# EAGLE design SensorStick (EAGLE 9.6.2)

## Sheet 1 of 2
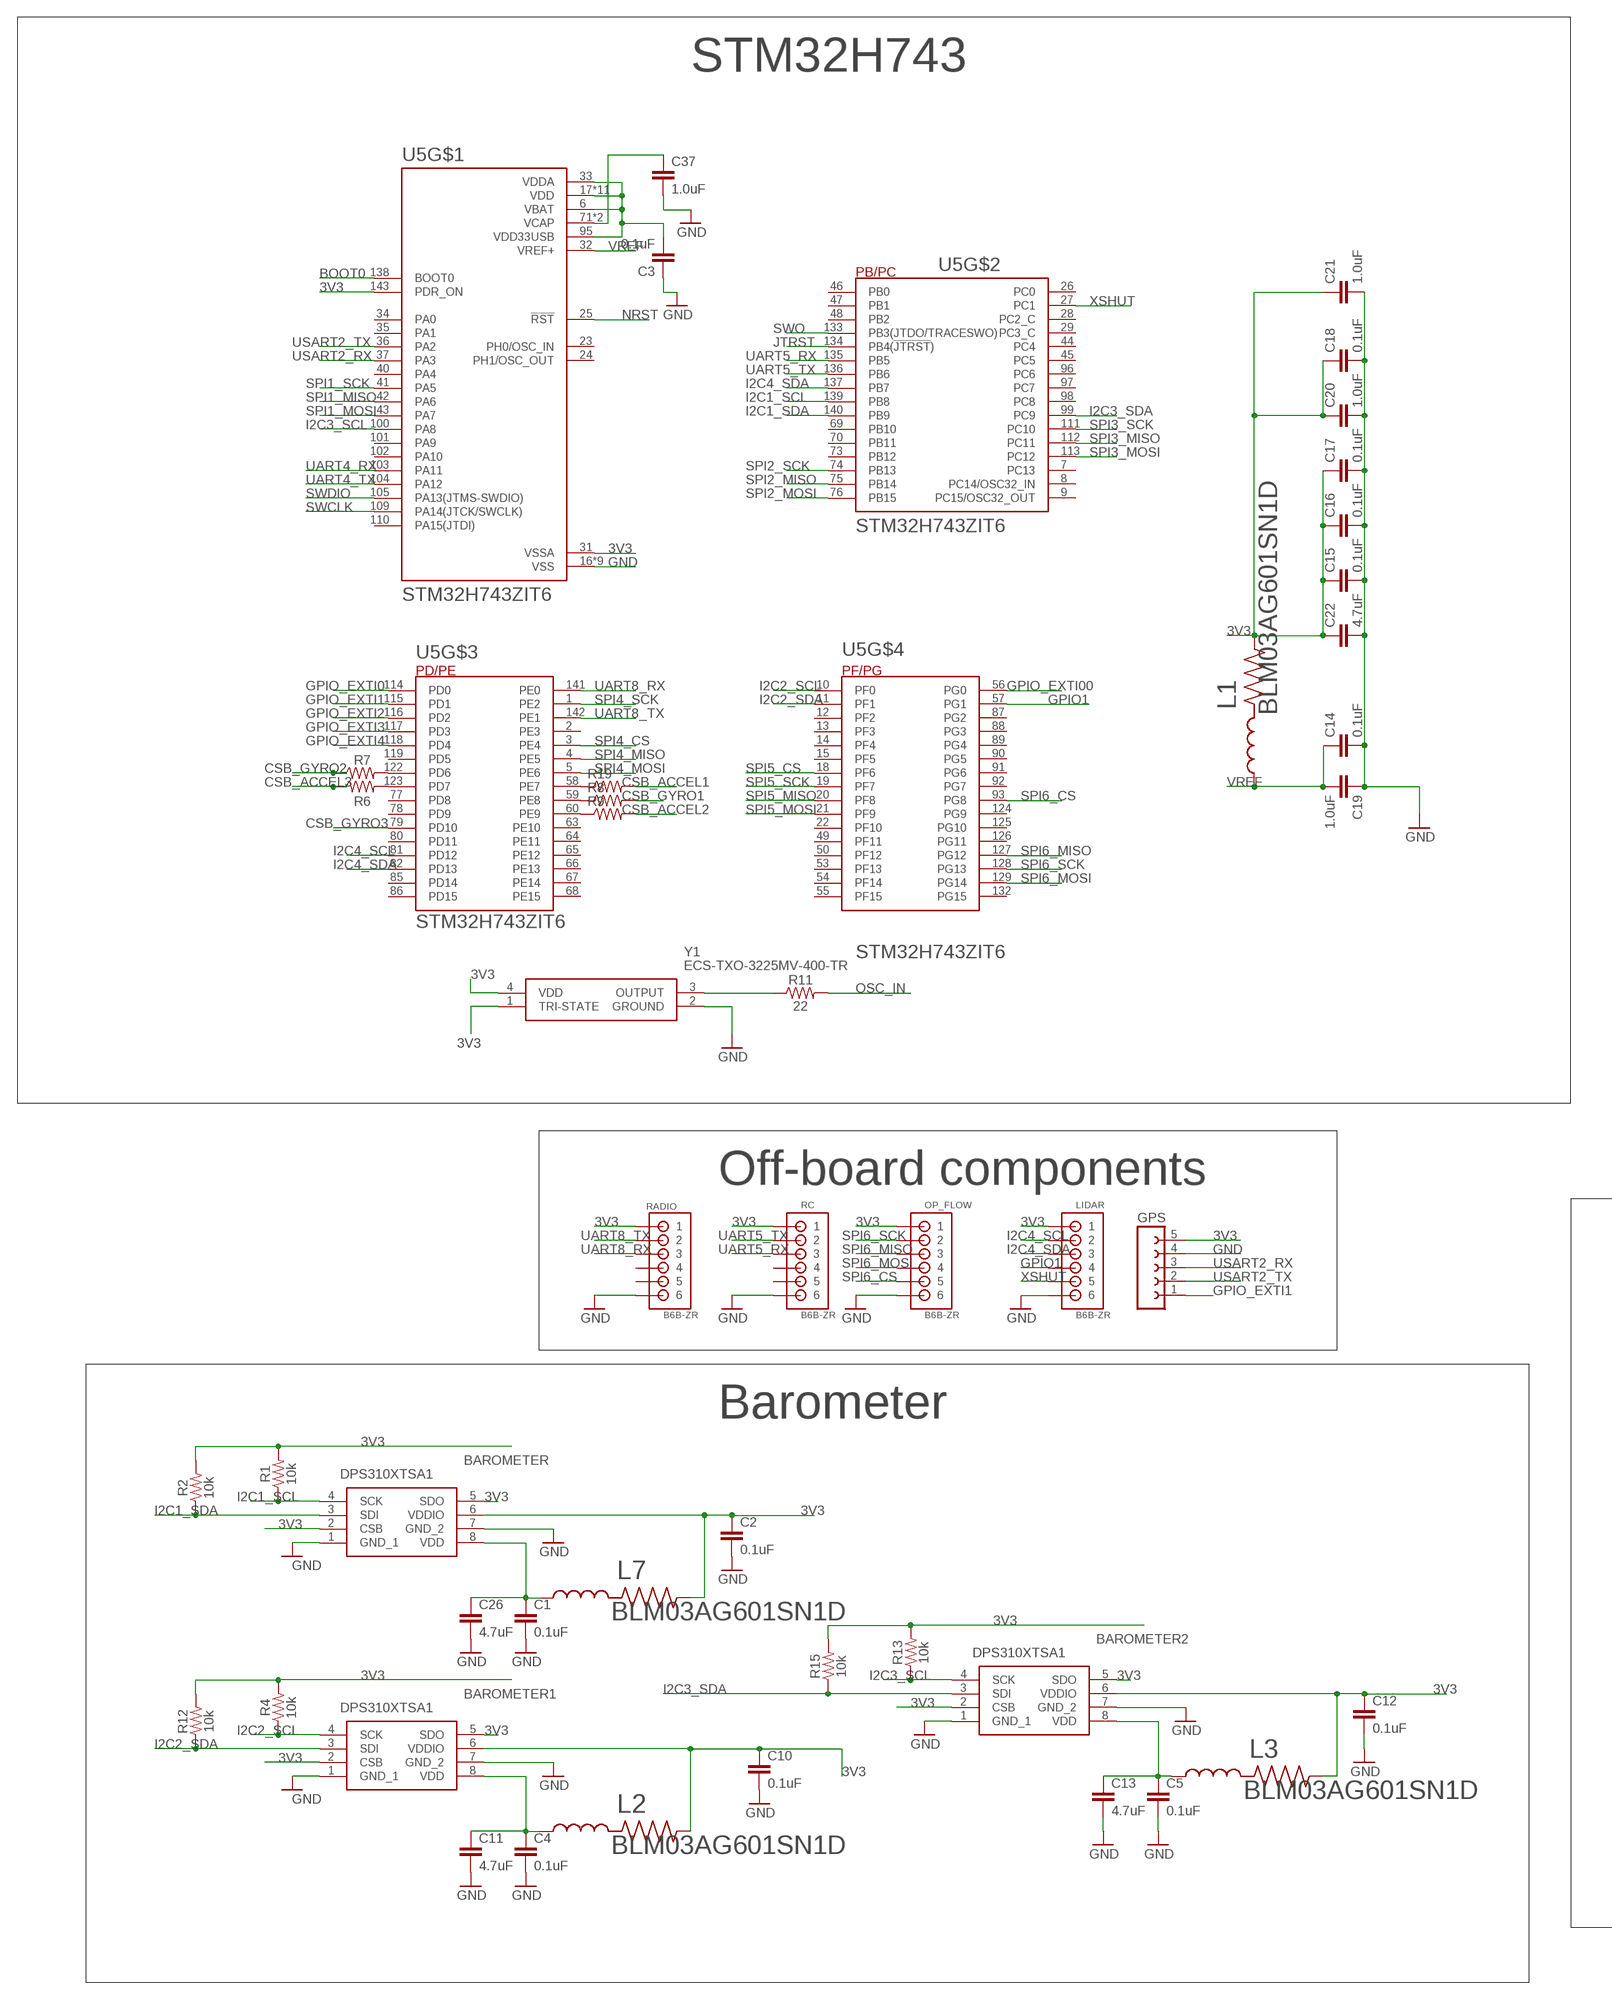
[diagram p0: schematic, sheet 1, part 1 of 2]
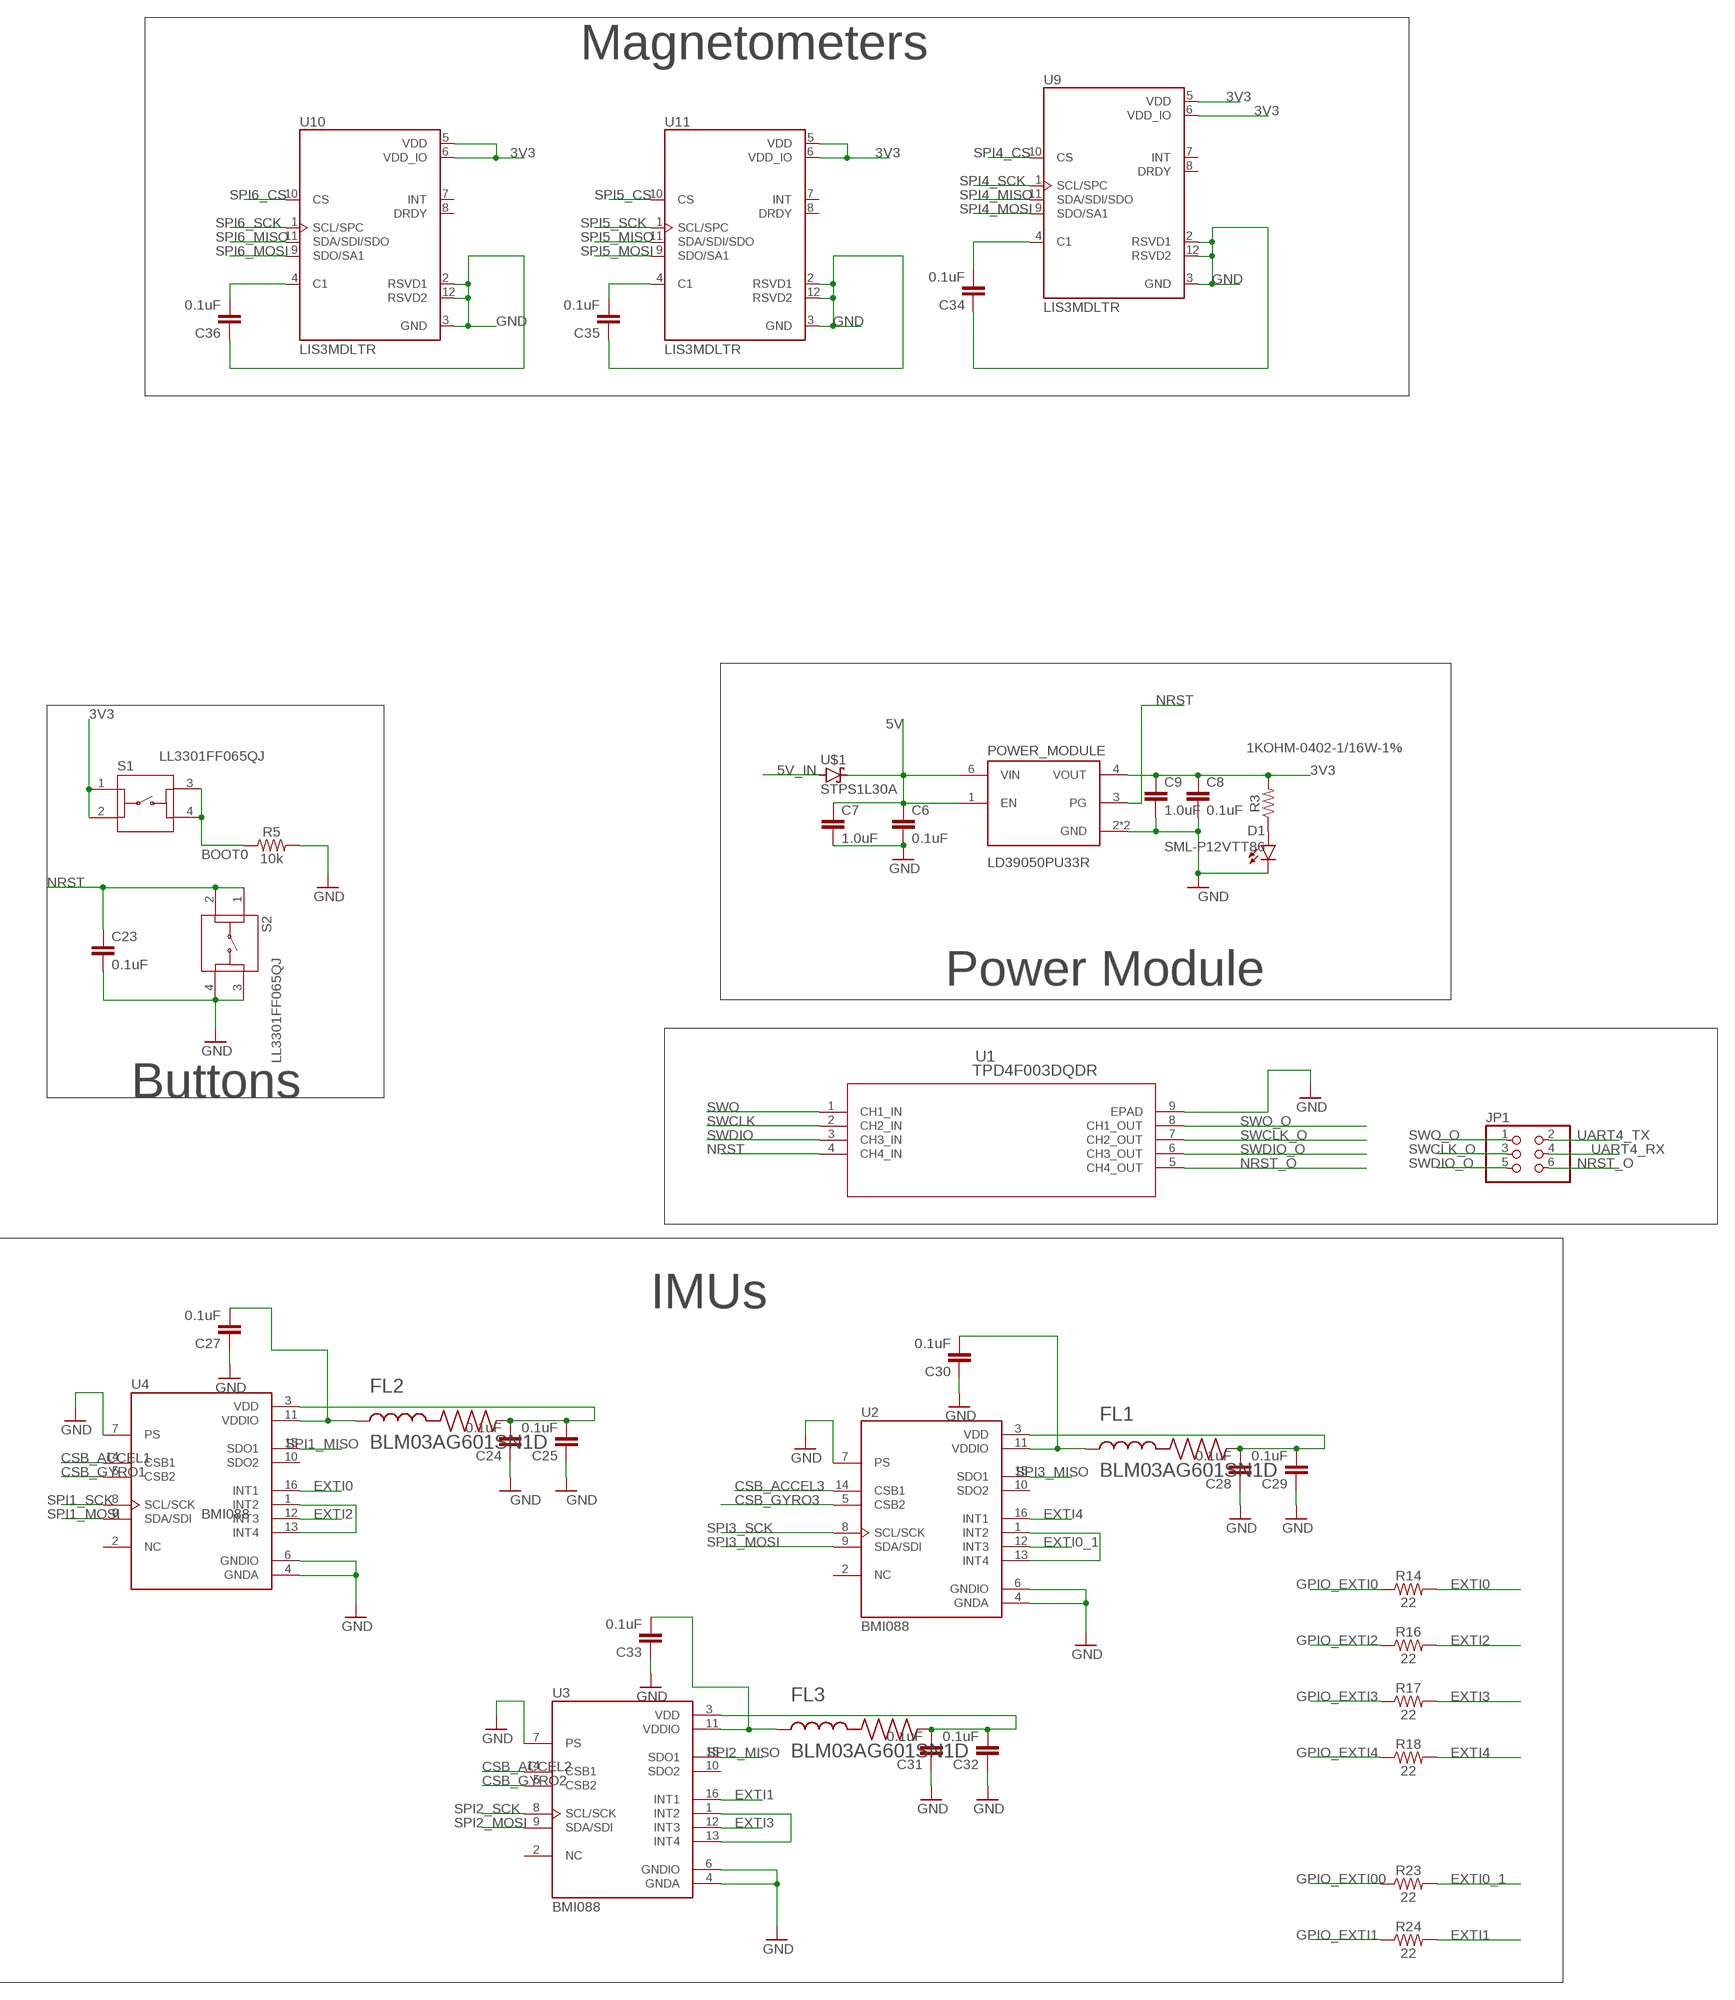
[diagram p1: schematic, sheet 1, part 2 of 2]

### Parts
BAROMETER  DPS310XTSA1  [DPS310XTSA1]
BAROMETER1  DPS310XTSA1  [DPS310XTSA1]
BAROMETER2  DPS310XTSA1  [DPS310XTSA1]
C1  0.1uF  0.1UF-0402-6.3V-10%-X7R  [0402]
C2  0.1uF  0.1UF-0402-6.3V-10%-X7R  [0402]
C3  0.1uF  0.1UF-0603-25V-5%  [0603]
C4  0.1uF  0.1UF-0402-6.3V-10%-X7R  [0402]
C5  0.1uF  0.1UF-0402-6.3V-10%-X7R  [0402]
C6  0.1uF  0.1UF-0402-6.3V-10%-X7R  [0402]
C7  1.0uF  1.0UF-0402-16V-10%  [0402]
C8  0.1uF  0.1UF-0402-6.3V-10%-X7R  [0402]
C9  1.0uF  1.0UF-0402-16V-10%  [0402]
C10  0.1uF  0.1UF-0402-6.3V-10%-X7R  [0402]
C11  4.7uF  4.7UF0603  [0603]
C12  0.1uF  0.1UF-0402-6.3V-10%-X7R  [0402]
C13  4.7uF  4.7UF0603  [0603]
C14  0.1uF  0.1UF-0603-25V-5%  [0603]
C15  0.1uF  0.1UF-0603-25V-5%  [0603]
C16  0.1uF  0.1UF-0603-25V-5%  [0603]
C17  0.1uF  0.1UF-0603-25V-5%  [0603]
C18  0.1uF  0.1UF-0603-25V-5%  [0603]
C19  1.0uF  1.0UF-0805-25V-10%  [0805]
C20  1.0uF  1.0UF-0805-25V-10%  [0805]
C21  1.0uF  1.0UF-0805-25V-10%  [0805]
C22  4.7uF  4.7UF0603  [0603]
C23  0.1uF  0.1UF-0603-25V-5%  [0603]
C24  0.1uF  0.1UF-0603-25V-5%  [0603]
C25  0.1uF  0.1UF-0603-25V-5%  [0603]
C26  4.7uF  4.7UF0603  [0603]
C27  0.1uF  0.1UF-0603-25V-5%  [0603]
C28  0.1uF  0.1UF-0603-25V-5%  [0603]
C29  0.1uF  0.1UF-0603-25V-5%  [0603]
C30  0.1uF  0.1UF-0603-25V-5%  [0603]
C31  0.1uF  0.1UF-0603-25V-5%  [0603]
C32  0.1uF  0.1UF-0603-25V-5%  [0603]
C33  0.1uF  0.1UF-0603-25V-5%  [0603]
C34  0.1uF  0.1UF-0603-25V-5%  [0603]
C35  0.1uF  0.1UF-0603-25V-5%  [0603]
C36  0.1uF  0.1UF-0603-25V-5%  [0603]
C37  1.0uF  1.0UF-0805-25V-10%  [0805]
D1  SML-P12VTT86  [LED_SML-P11UTT86R]
FL1  BLM03AG601SN1D  [BEADC0603X33N]
FL2  BLM03AG601SN1D  [BEADC0603X33N]
FL3  BLM03AG601SN1D  [BEADC0603X33N]
GPS  FE05-1  [FE05-1]
JP1  PINHD-2X3  [2X03]
L1  BLM03AG601SN1D  [BEADC0603X33N]
L2  BLM03AG601SN1D  [BEADC0603X33N]
L3  BLM03AG601SN1D  [BEADC0603X33N]
L7  BLM03AG601SN1D  [BEADC0603X33N]
LIDAR  B6B-ZR  [B6B-ZR]
OP_FLOW  B6B-ZR  [B6B-ZR]
POWER_MODULE  LD39050PU33R  [SON95P300X300X100-7N]
R1  10k  10KOHM-0402-1/16W-1%  [0402]
R2  10k  10KOHM-0402-1/16W-1%  [0402]
R3  1KOHM-0402-1/16W-1%  [0402]
R4  10k  10KOHM-0402-1/16W-1%  [0402]
R5  10k  10KOHM-0603-1/10W-1%  [0603]
R6  RT0402FRE07220RL  [RESC1005X35N]
R7  RT0402FRE07220RL  [RESC1005X35N]
R8  RT0402FRE07220RL  [RESC1005X35N]
R9  RT0402FRE07220RL  [RESC1005X35N]
R11  22  22OHM-0402-1/10W-1%  [0402]
R12  10k  10KOHM-0402-1/16W-1%  [0402]
R13  10k  10KOHM-0402-1/16W-1%  [0402]
R14  22  22OHM-0402-1/10W-1%  [0402]
R15  10k  10KOHM-0402-1/16W-1%  [0402]
R16  22  22OHM-0402-1/10W-1%  [0402]
R17  22  22OHM-0402-1/10W-1%  [0402]
R18  22  22OHM-0402-1/10W-1%  [0402]
R19  RT0402FRE07220RL  [RESC1005X35N]
R23  22  22OHM-0402-1/10W-1%  [0402]
R24  22  22OHM-0402-1/10W-1%  [0402]
RADIO  B6B-ZR  [B6B-ZR]
RC  B6B-ZR  [B6B-ZR]
S1  LL3301FF065QJ  [LL3301FF065QJ]
S2  LL3301FF065QJ  [LL3301FF065QJ]
U1  TPD4F003DQDR  [DQD8_1P2X0P4]
U2  BMI088  [PQFN50P450X300X100-16N]
U3  BMI088  [PQFN50P450X300X100-16N]
U4  BMI088  [PQFN50P450X300X100-16N]
U5  STM32H743ZIT6  [QFP50P2200X2200X160-144N]
U9  LIS3MDLTR  [XDCR_LIS3MDLTR]
U10  LIS3MDLTR  [XDCR_LIS3MDLTR]
U11  LIS3MDLTR  [XDCR_LIS3MDLTR]
U$1  STPS1L30A  [DIOM5226X223N]
Y1  ECS-TXO-3225MV-400-TR  [ECSTXO3225MV400TR]

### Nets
3V2: C28.2 C29.2 FL1.2 U2.3(VDD)
3V3: BAROMETER1.2(CSB) BAROMETER1.5(SDO) BAROMETER1.6(VDDIO) BAROMETER2.2(CSB) BAROMETER2.5(SDO) BAROMETER2.6(VDDIO) BAROMETER.2(CSB) BAROMETER.5(SDO) BAROMETER.6(VDDIO) C2.1 C3.2 C8.1 C9.1 C10.1 C12.1 C15.1 C16.1 C17.1 C18.1 C20.1 C21.1 C22.1 GPS.5 L1.2 L2.2 L3.2 L7.2 LIDAR.1 OP_FLOW.1 POWER_MODULE.4(VOUT) R1.2 R2.2 R3.2 R4.2 R12.2 R13.2 R15.2 RADIO.1 RC.1 S1.1 S1.2 U5.6(VBAT) U5.17(VDD) U5.30(VDD) U5.31(VSSA) U5.33(VDDA) U5.39(VDD) U5.52(VDD) U5.62(VDD) U5.72(VDD) U5.84(VDD) U5.95(VDD33USB) U5.108(VDD) U5.121(VDD) U5.131(VDD) U5.143(PDR_ON) U5.144(VDD) U9.5(VDD) U9.6(VDD_IO) U10.5(VDD) U10.6(VDD_IO) U11.5(VDD) U11.6(VDD_IO) Y1.1(TRI-STATE) Y1.4(VDD)
3V4: C24.2 C25.2 FL2.2 U4.3(VDD)
3V5: C31.2 C32.2 FL3.2 U3.3(VDD)
5V: C6.1 C7.1 POWER_MODULE.1(EN) POWER_MODULE.6(VIN) U$1.1(C)
5V_IN: U$1.2(A)
BOOT0: R5.1 S1.3 S1.4 U5.138(BOOT0)
CSB_ACCEL1: R19.2 U4.14(CSB1)
CSB_ACCEL2: R9.2 U3.14(CSB1)
CSB_ACCEL3: R6.1 U2.14(CSB1)
CSB_GYRO1: R8.2 U4.5(CSB2)
CSB_GYRO2: R7.1 U3.5(CSB2)
CSB_GYRO3: U2.5(CSB2) U5.79(PD10)
EXTI0: R14.2 U4.16(INT1)
EXTI0_1: R23.2 U2.12(INT3)
EXTI1: R24.2 U3.16(INT1)
EXTI2: R16.2 U4.12(INT3)
EXTI3: R17.2 U3.12(INT3)
EXTI4: R18.2 U2.16(INT1)
GND: BAROMETER1.1(GND_1) BAROMETER1.7(GND_2) BAROMETER2.1(GND_1) BAROMETER2.7(GND_2) BAROMETER.1(GND_1) BAROMETER.7(GND_2) C1.2 C2.2 C3.1 C4.2 C5.2 C6.2 C7.2 C8.2 C9.2 C10.2 C11.2 C12.2 C13.2 C14.2 C15.2 C16.2 C17.2 C18.2 C19.1 C20.2 C21.2 C22.2 C23.2 C24.1 C25.1 C26.2 C27.1 C28.1 C29.1 C30.1 C31.1 C32.1 C33.1 C34.1 C35.1 C36.1 C37.2 D1.C GPS.4 LIDAR.6 OP_FLOW.6 POWER_MODULE.2(GND) POWER_MODULE.7(GND) R5.2 S2.3 S2.4 U1.9(EPAD) U2.4(GNDA) U2.6(GNDIO) U2.7(PS) U3.4(GNDA) U3.6(GNDIO) U3.7(PS) U4.4(GNDA) U4.6(GNDIO) U4.7(PS) U5.16(VSS) U5.38(VSS) U5.51(VSS) U5.61(VSS) U5.83(VSS) U5.94(VSS) U5.107(VSS) U5.120(VSS) U5.130(VSS) U9.2(RSVD1) U9.3(GND) U9.12(RSVD2) U10.2(RSVD1) U10.3(GND) U10.12(RSVD2) U11.2(RSVD1) U11.3(GND) U11.12(RSVD2) Y1.2(GROUND)
GPIO1: LIDAR.4 U5.57(PG1)
GPIO_EXTI0: R14.1 U5.114(PD0)
GPIO_EXTI00: R23.1 U5.56(PG0)
GPIO_EXTI1: GPS.1 R24.1 U5.115(PD1)
GPIO_EXTI2: R16.1 U5.116(PD2)
GPIO_EXTI3: R17.1 U5.117(PD3)
GPIO_EXTI4: R18.1 U5.118(PD4)
I2C1_SCL: BAROMETER.4(SCK) R1.1 U5.139(PB8)
I2C1_SDA: BAROMETER.3(SDI) R2.1 U5.140(PB9)
I2C2_SCL: BAROMETER1.4(SCK) R4.1 U5.10(PF0)
I2C2_SDA: BAROMETER1.3(SDI) R12.1 U5.11(PF1)
I2C3_SCL: BAROMETER2.4(SCK) R13.1 U5.100(PA8)
I2C3_SDA: BAROMETER2.3(SDI) R15.1 U5.99(PC9)
I2C4_SCL: LIDAR.2 U5.81(PD12)
I2C4_SDA: LIDAR.3 U5.82(PD13) U5.137(PB7)
IMU_INT3: U3.1(INT2) U3.13(INT4)
JTRST: U5.134(PB4(!JTRST!))
N$1: R11.1 Y1.3(OUTPUT)
N$2: BAROMETER2.8(VDD) C5.1 C13.1 L3.1
N$3: BAROMETER1.8(VDD) C4.1 C11.1 L2.1
N$4: C34.2 U9.4(C1)
N$5: D1.A R3.1
N$6: BAROMETER.8(VDD) C1.1 C26.1 L7.1
N$7: C35.2 U11.4(C1)
N$8: C27.2 FL2.1 U4.11(VDDIO)
N$9: C30.2 FL1.1 U2.11(VDDIO)
N$10: C33.2 FL3.1 U3.11(VDDIO)
N$11: C36.2 U10.4(C1)
N$12: C37.1 U5.71(VCAP) U5.106(VCAP)
N$13: R6.2 U5.123(PD7)
N$14: R7.2 U5.122(PD6)
N$15: R19.1 U5.58(PE7)
N$16: R8.1 U5.59(PE8)
N$17: R9.1 U5.60(PE9)
N$19: RADIO.6 RC.6 ; supply symbol labelled GND
N$20: U4.1(INT2) U4.13(INT4)
N$23: U2.1(INT2) U2.13(INT4)
NRST: C23.1 POWER_MODULE.3(PG) S2.1 S2.2 U1.4(CH4_IN) U5.25(!RST)
NRST_O: JP1.6 U1.5(CH4_OUT)
OSC_IN: R11.2
SPI1_MISO: U4.15(SDO1) U5.42(PA6)
SPI1_MOSI: U4.9(SDA/SDI) U5.43(PA7)
SPI1_SCK: U4.8(SCL/SCK) U5.41(PA5)
SPI2_MISO: U3.15(SDO1) U5.75(PB14)
SPI2_MOSI: U3.9(SDA/SDI) U5.76(PB15)
SPI2_SCK: U3.8(SCL/SCK) U5.74(PB13)
SPI3_MISO: U2.15(SDO1) U5.112(PC11)
SPI3_MOSI: U2.9(SDA/SDI) U5.113(PC12)
SPI3_SCK: U2.8(SCL/SCK) U5.111(PC10)
SPI4_CS: U5.3(PE4) U9.10(CS)
SPI4_MISO: U5.4(PE5) U9.11(SDA/SDI/SDO)
SPI4_MOSI: U5.5(PE6) U9.9(SDO/SA1)
SPI4_SCK: U5.1(PE2) U9.1(SCL/SPC)
SPI5_CS: U5.18(PF6) U11.10(CS)
SPI5_MISO: U5.20(PF8) U11.11(SDA/SDI/SDO)
SPI5_MOSI: U5.21(PF9) U11.9(SDO/SA1)
SPI5_SCK: U5.19(PF7) U11.1(SCL/SPC)
SPI6_CS: OP_FLOW.5 U5.93(PG8) U10.10(CS)
SPI6_MISO: OP_FLOW.3 U5.127(PG12) U10.11(SDA/SDI/SDO)
SPI6_MOSI: OP_FLOW.4 U5.129(PG14) U10.9(SDO/SA1)
SPI6_SCK: OP_FLOW.2 U5.128(PG13) U10.1(SCL/SPC)
SWCLK: U1.2(CH2_IN) U5.109(PA14(JTCK/SWCLK))
SWCLK_O: JP1.3 U1.7(CH2_OUT)
SWDIO: U1.3(CH3_IN) U5.105(PA13(JTMS-SWDIO))
SWDIO_O: JP1.5 U1.6(CH3_OUT)
SWO: U1.1(CH1_IN) U5.133(PB3(JTDO/TRACESWO))
SWO_O: JP1.1 U1.8(CH1_OUT)
UART4_RX: JP1.4 U5.103(PA11)
UART4_TX: JP1.2 U5.104(PA12)
UART5_RX: RC.3 U5.135(PB5)
UART5_TX: RC.2 U5.136(PB6)
UART8_RX: RADIO.3 U5.141(PE0)
UART8_TX: RADIO.2 U5.142(PE1)
USART2_RX: GPS.3 U5.37(PA3)
USART2_TX: GPS.2 U5.36(PA2)
VREF: C14.1 C19.2 L1.1 U5.32(VREF+)
XSHUT: LIDAR.5 U5.27(PC1)
Unconnected: RADIO.4 RADIO.5 RC.4 RC.5 U2.2(NC) U2.10(SDO2) U3.2(NC) U3.10(SDO2) U4.2(NC) U4.10(SDO2) U5.2(PE3) U5.7(PC13) U5.8(PC14/OSC32_IN) U5.9(PC15/OSC32_OUT) U5.12(PF2) U5.13(PF3) U5.14(PF4) U5.15(PF5) U5.22(PF10) U5.23(PH0/OSC_IN) U5.24(PH1/OSC_OUT) U5.26(PC0) U5.28(PC2_C) U5.29(PC3_C) U5.34(PA0) U5.35(PA1) U5.40(PA4) U5.44(PC4) U5.45(PC5) U5.46(PB0) U5.47(PB1) U5.48(PB2) U5.49(PF11) U5.50(PF12) U5.53(PF13) U5.54(PF14) U5.55(PF15) U5.63(PE10) U5.64(PE11) U5.65(PE12) U5.66(PE13) U5.67(PE14) U5.68(PE15) U5.69(PB10) U5.70(PB11) U5.73(PB12) U5.77(PD8) U5.78(PD9) U5.80(PD11) U5.85(PD14) U5.86(PD15) U5.87(PG2) U5.88(PG3) U5.89(PG4) U5.90(PG5) U5.91(PG6) U5.92(PG7) U5.96(PC6) U5.97(PC7) U5.98(PC8) U5.101(PA9) U5.102(PA10) U5.110(PA15(JTDI)) U5.119(PD5) U5.124(PG9) U5.125(PG10) U5.126(PG11) U5.132(PG15) U9.7(INT) U9.8(DRDY) U10.7(INT) U10.8(DRDY) U11.7(INT) U11.8(DRDY)

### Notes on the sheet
- Magnetometers
- STM32H743
- Power Module
- Buttons
- Off-board components
- IMUs
- Barometer

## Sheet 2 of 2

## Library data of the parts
BAROMETER BAROMETER1 BAROMETER2 = DPS310XTSA1:DPS310XTSA1: INFINEON - DPS310XTSA1 - DIGITAL PRESSURE SENSOR, 1200HPA, VLGA-8 Source: Datasheet; ARROW_PART_NUMBER: DPS310XTSA1; ARROW_PRICE-STOCK: https://www.arrow.com/en/products/dps310xtsa1/infineon-technologies-ag?region=nac; DESCRIPTION: INFINEON - DPS310XTSA1 - DIGITAL PRESSURE SENSOR, 1200HPA, VLGA-8; HEIGHT: 1.01mm; MANUFACTURER_NAME: Infineon; MANUFACTURER_PART_NUMBER: DPS310XTSA1; MOUSER_PART_NUMBER: 726-DPS310XTSA1; MOUSER_PRICE-STOCK: https://www.mouser.co.uk/ProductDetail/Infineon-Technologies/DPS310XTSA1?qs=uuTTuBTXn66Ynca8WHwycg%3D%3D
C1 C2 C4-C6 C8 C10 C12 = SparkFun-Capacitors:0.1UF: 0.1µF ceramic capacitors; PROD_ID: CAP-14993
C3 C14-C18 C23-C25 C27-C36 = SparkFun-Capacitors:0.1UF: 0.1µF ceramic capacitors; PROD_ID: CAP-08604
C7 C9 = SparkFun-Capacitors:1.0UF: 1µF ceramic capacitors; PROD_ID: CAP-12417
C11 C13 C22 C26 = SparkFun-Capacitors:4.7UF: 4.7µF ceramic capacitors; PROD_ID: CAP-08280
C19-C21 C37 = SparkFun-Capacitors:1.0UF: 1µF ceramic capacitors; PROD_ID: CAP-08064
D1 = ce-capstone:SML-P12VTT86: SML-P1 Series Red 0402 Clear 60 mcd 2 V Surface Mount PICOLED LED; AVAILABILITY: Unavailable; DESCRIPTION: Red 630nm LED Indication - Discrete 2V 0402 _1006 Metric_; MF: Rohm; MP: SML-P12VTT86; PACKAGE: 0402 Rohm; PRICE: None
FL1-FL3 L1-L3 L7 = BLM03AG601SN1D:BLM03AG601SN1D: Ferrite Bead 600R 100mA SMD 0201 Check availability; AVAILABILITY: In Stock; CHECK_PRICES: https://www.snapeda.com/parts/BLM03AG601SN1D/Murata/view-part/?ref=eda; DESCRIPTION: 600 Ohms @ 100 MHz 1 - Ferrite Bead 0201 (0603 Metric) 100mA 1.5Ohm; MF: Murata Electronics; MP: BLM03AG601SN1D; PACKAGE: 0603 Murata; PRICE: None; PURCHASE-URL: https://www.snapeda.com/api/url_track_click_mouser/?unipart_id=283112&manufacturer=Murata Electronics&part_name=BLM03AG601SN1D&search_term=None; SNAPEDA_LINK: https://www.snapeda.com/parts/BLM03AG601SN1D/Murata/view-part/?ref=snap
GPS = con-lsta:FE05-1: FEMALE HEADER; OC_FARNELL: unknown; OC_NEWARK: unknown
JP1 = pinhead:PINHD-2X3: PIN HEADER
LIDAR OP_FLOW RADIO RC = jst:B6B-ZR: JST-ZH Connector 6 pol, 1.5mm pitch Package: B6B-ZR Source: http://www.jst-mfg.com/product/pdf/eng/eZH.pdf
POWER_MODULE = ce-capstone:LD39050PU33R: LD39050 Series 500 mA 3.3 V Fixed Low Noise LDO Voltage Regulator - DFN-6; AVAILABILITY: Unavailable; DESCRIPTION: Linear Voltage Regulator IC 1 Output 500mA 6-DFN _3x3_; MF: STMicroelectronics; MP: LD39050PU33R; PACKAGE: DFN-6 STMicroelectronics; PRICE: None
R1 R2 R4 R12 R13 R15 = SparkFun-Resistors:10KOHM: 10kΩ resistor; PROD_ID: RES-14241
R3 = SparkFun-Resistors:1KOHM: 1kΩ resistor; PROD_ID: RES-14342
R5 = SparkFun-Resistors:10KOHM: 10kΩ resistor; PROD_ID: RES-00824
R6-R9 R19 = ce-capstone:RT0402FRE07220RL: RES SMD 4.7K OHM 1% 1/16W 0402; DESCRIPTION: 4.7 kOhms ±1% 0.063W, 1/16W Chip Resistor 0402 _1005 Metric_ Thin Film; DIGI-KEY_PART_NUMBER: YAG3347CT-ND; DIGI-KEY_PURCHASE_URL: https://www.digikey.com/product-detail/en/yageo/RT0402FRE074K7L/YAG3347CT-ND/5418052?utm_source=snapeda&utm_medium=aggregator&utm_campaign=symbol; MF: Yageo; MP: RT0402FRE074K7L; PACKAGE: 1005 Yageo
R11 R14 R16-R18 R23 R24 = SparkFun-Resistors:22OHM: 22Ω resistor; PROD_ID: RES-12427
S1 S2 = ce-capstone:LL3301FF065QJ: Pushbutton Switches 50mA 12VDC F065 7.0mm J-Lead Source: Datasheet; DESCRIPTION: Pushbutton Switches 50mA 12VDC F065 7.0mm J-Lead; HEIGHT: 7.3mm; MANUFACTURER_NAME: E-Switch; MANUFACTURER_PART_NUMBER: LL3301FF065QJ; MOUSER_PART_NUMBER: 612-LL3301FF065QJ; MOUSER_PRICE-STOCK: https://www.mouser.com/Search/Refine.aspx?Keyword=612-LL3301FF065QJ
U1 = TPD4F003DQDR:TPD4F003DQDR; COPYRIGHT: Copyright (C) 2023 Ultra Librarian. All rights reserved.; DIGI-KEY_PART_NUMBER_1: 296-25817-1-ND; DIGI-KEY_PART_NUMBER_2: 296-25817-2-ND; DIGI-KEY_PART_NUMBER_3: 296-25817-6-ND; DIGI-KEY_PART_NUMBER_4: 2156-TPD4F003DQDR-ND; MANUFACTURER_PART_NUMBER: TPD4F003DQDR; MFR_NAME: Texas Instruments
U2-U4 = BMI088:BMI088: High-performance 6-axis inertial sensor (accelerometer + gyroscope) Check prices Check availability; AVAILABILITY: In Stock; CHECK_PRICES: https://www.snapeda.com/parts/BMI088/Bosch+Sensortec/view-part/?ref=eda; DESCRIPTION: Accelerometer, Gyroscope, 6 Axis Sensor I2C, SPI Output; MF: Bosch Sensortec; MP: BMI088; PACKAGE: VFLGA-16 Bosch Sensortec; PRICE: None; PURCHASE-URL: https://www.snapeda.com/api/url_track_click_mouser/?unipart_id=2774026&manufacturer=Bosch Sensortec&part_name=BMI088&search_term=None; SNAPEDA_LINK: https://www.snapeda.com/parts/BMI088/Bosch+Sensortec/view-part/?ref=snap
U5 = STM32H743ZIT6:STM32H743ZIT6: High-performance and DSP with DP-FPU, ARM Cortex-M7 MCU with 2MBytes Flash, 1MB RAM, 400 MHz CPU, Art Accelerator, L1... Check availability; AVAILABILITY: In Stock; CHECK_PRICES: https://www.snapeda.com/parts/STM32H743ZIT6/STMicroelectronics/view-part/?ref=eda; DESCRIPTION: ARM® Cortex®-M7 STM32H7 Microcontroller IC 32-Bit Single-Core 480MHz 2MB (2M x 8) FLASH 144-LQFP (20x20); MF: STMicroelectronics; MP: STM32H743ZIT6; PACKAGE: LQFP-144 STMicroelectronics; PRICE: None; PURCHASE-URL: https://www.snapeda.com/api/url_track_click_mouser/?unipart_id=1041111&manufacturer=STMicroelectronics&part_name=STM32H743ZIT6&search_term=stm32h743; SNAPEDA_LINK: https://www.snapeda.com/parts/STM32H743ZIT6/STMicroelectronics/view-part/?ref=snap; SPICEPREFIX: X
U9-U11 = LIS3MDLTR:LIS3MDLTR: LIS3MDL Series 3 Axis ±2/±8/±12/±16 g 3.6V High Performance Magnetometer LGA-12 Check availability; AVAILABILITY: In Stock; CHECK_PRICES: https://www.snapeda.com/parts/LIS3MDLTR/STMicroelectronics/view-part/?ref=eda; DESCRIPTION: Magnetoresistive Sensor X, Y, Z Axis 12-LGA (2x2); MF: STMicroelectronics; MP: LIS3MDLTR; PACKAGE: VFLGA-12 STMicroelectronics; PRICE: None; PURCHASE-URL: https://www.snapeda.com/api/url_track_click_mouser/?unipart_id=382740&manufacturer=STMicroelectronics&part_name=LIS3MDLTR&search_term=None; SNAPEDA_LINK: https://www.snapeda.com/parts/LIS3MDLTR/STMicroelectronics/view-part/?ref=snap
U$1 = ce-capstone:STPS1L30A
Y1 = SamacSys_Parts:ECS-TXO-3225MV-400-TR: TCXO Oscillators 40.000 MHZ Multi-Volt +1.7 3.6V HCMOS TCXO +/-2.5 ppm -30 +85 C 3.2x 2.5mm RoHS Source: Datasheet; DESCRIPTION: TCXO Oscillators 40.000 MHZ Multi-Volt +1.7 3.6V HCMOS TCXO +/-2.5 ppm -30 +85 C 3.2x 2.5mm RoHS; HEIGHT: 1.2mm; MANUFACTURER_NAME: ECS; MANUFACTURER_PART_NUMBER: ECS-TXO-3225MV-400-TR

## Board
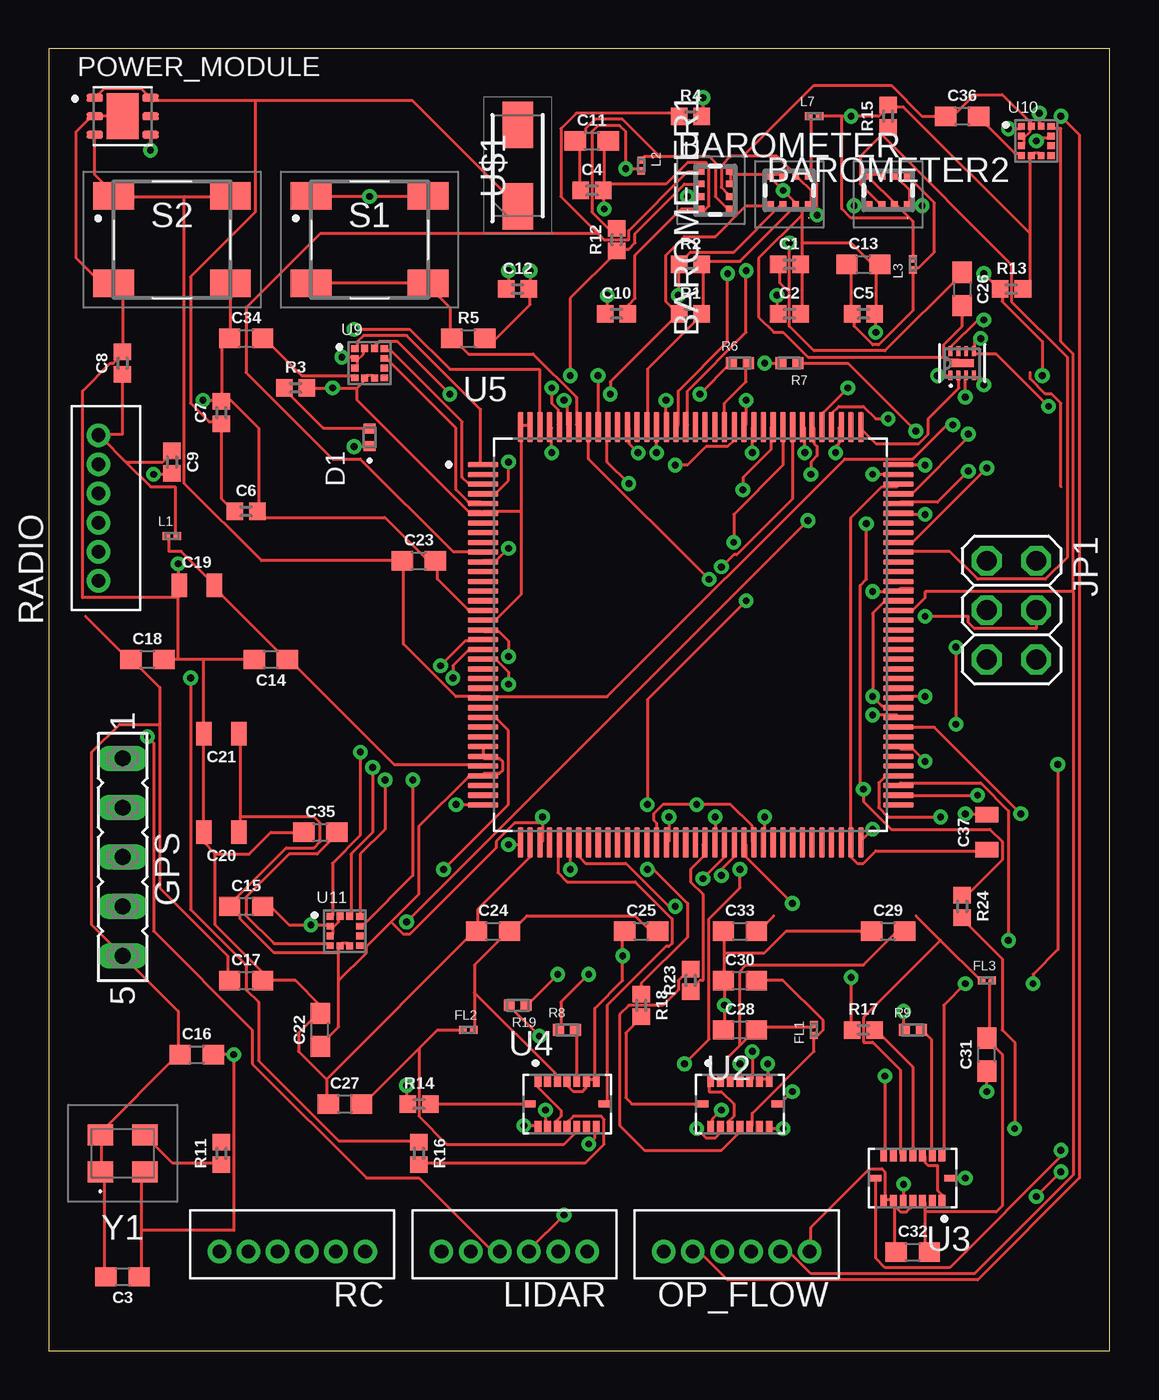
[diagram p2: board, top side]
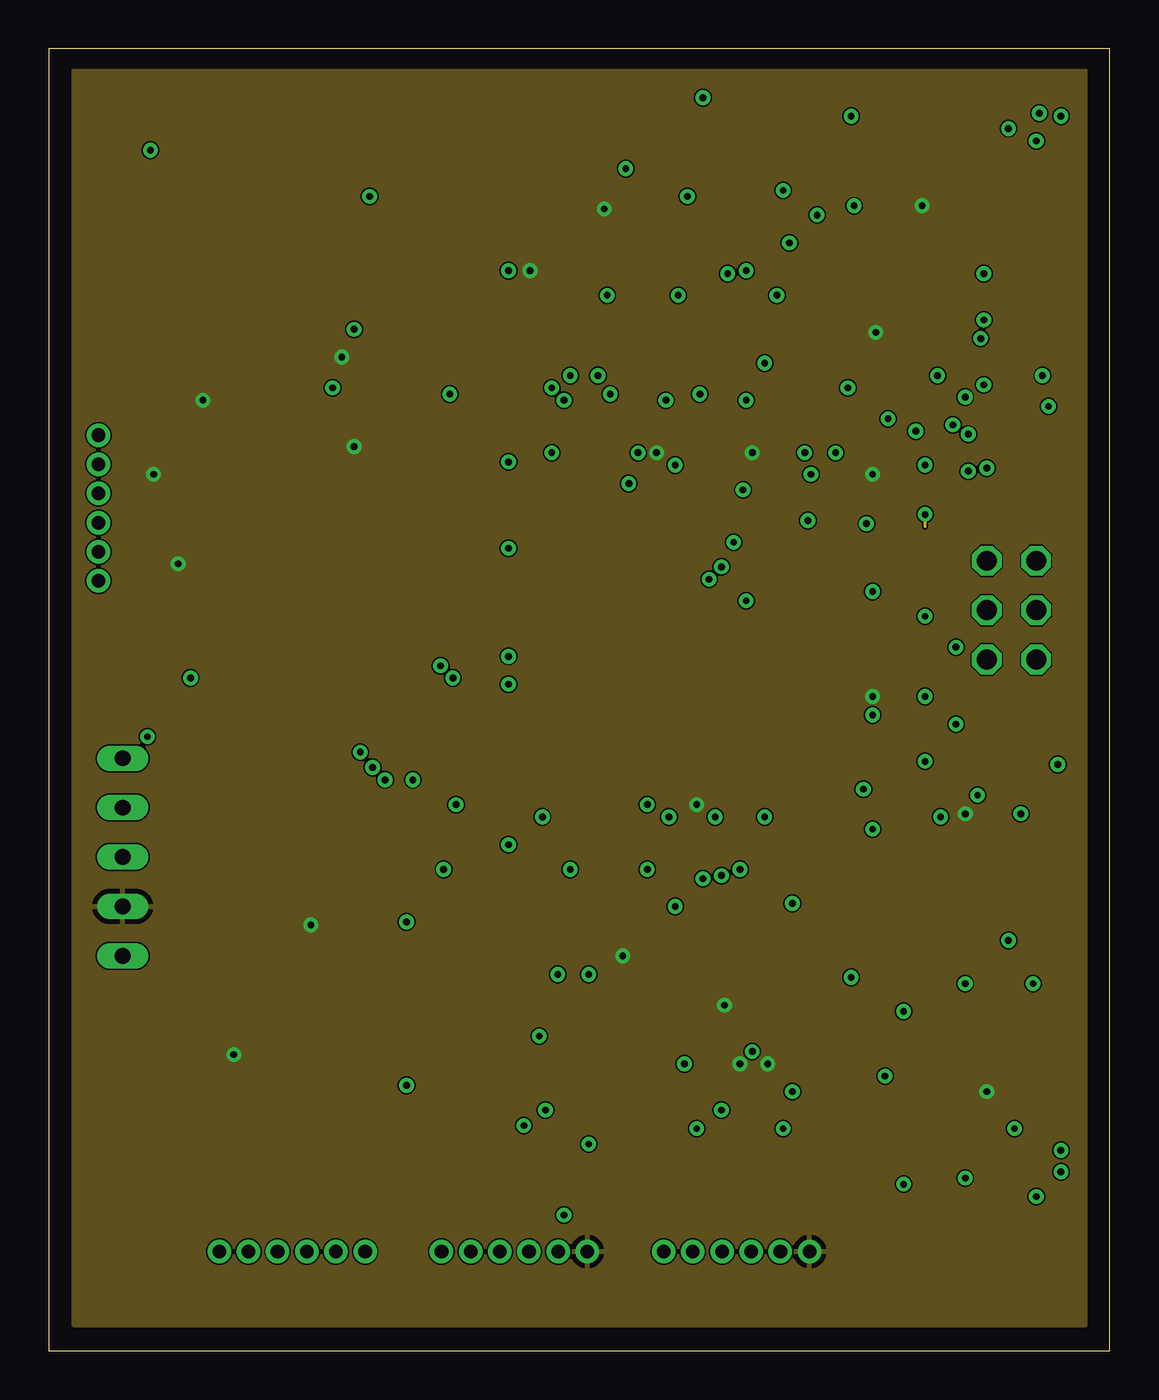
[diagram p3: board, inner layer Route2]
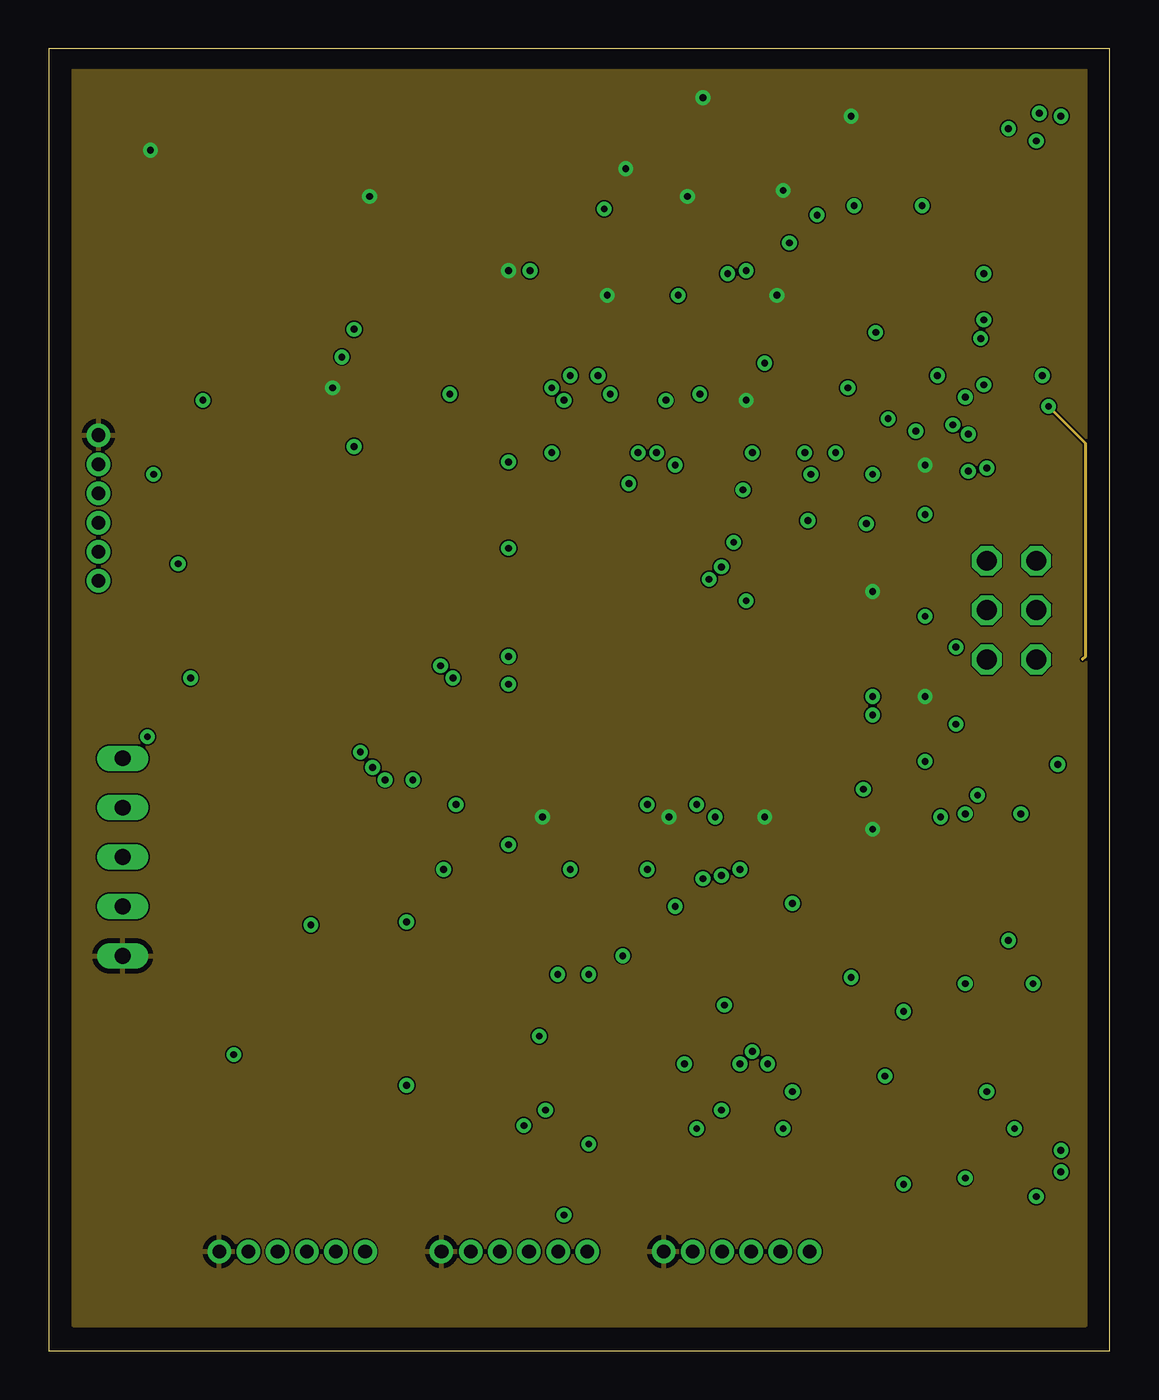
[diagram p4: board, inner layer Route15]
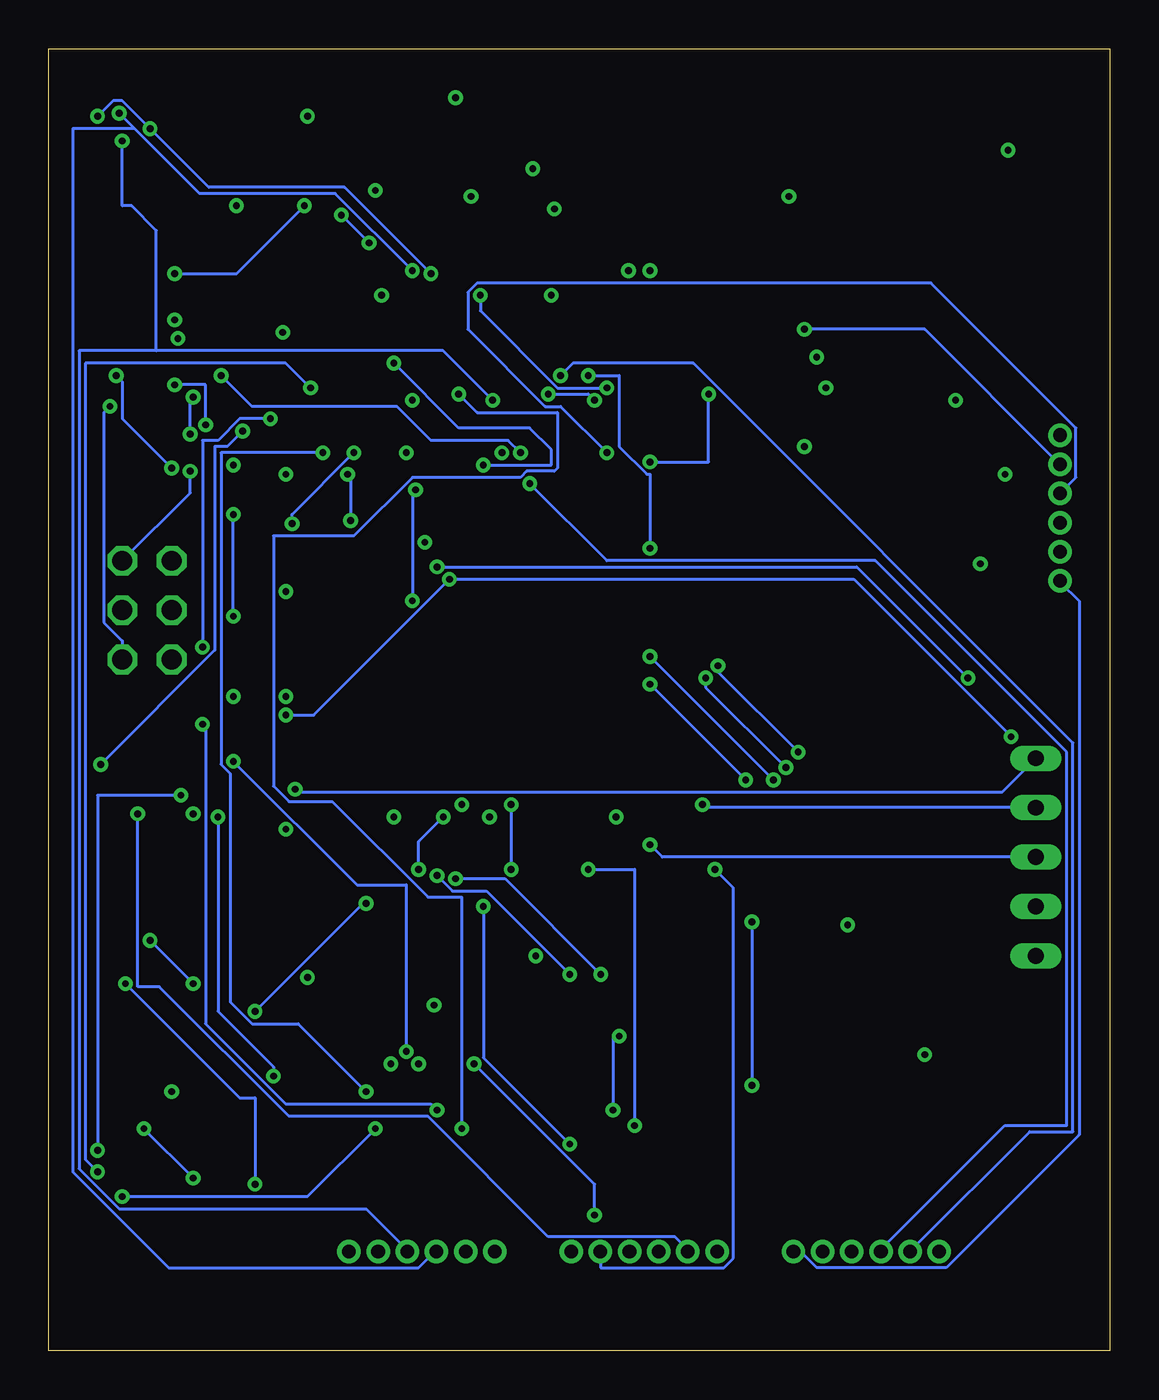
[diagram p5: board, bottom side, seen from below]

Size 54.59 x 66.98 mm. Coordinates in mm from the lower left corner, seen from the top.
Outline: 0,0 54.59,0 54.59,66.98 0,66.98 0,0
Copper layers (1+2*15+16): Top 0.035mm / dielectric 1.5mm / Route2 0.035mm / dielectric 0.15mm / Route15 0.035mm / dielectric 0.2mm / Bottom 0.035mm
Design rules "default *": minimum track width 6mil, minimum drill 0.35mm, track to track 3mil, track to pad 3mil, pad to pad 3mil, via to via 3mil, smd to smd 3mil, copper to edge 40mil, drill to drill 6mil, minimum pad ring 10mil, minimum via ring 8mil, stop-mask expansion 4mil, vias tented up to drill 0mil, thermal gap 10mil

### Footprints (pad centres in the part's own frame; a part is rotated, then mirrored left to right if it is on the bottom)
DPS310XTSA1 = smd 0.35 x 0.35: 1 0.975,-0.725; 2 0.325,-0.725; 3 -0.325,-0.725; 4 -0.975,-0.725; 5 -0.975,0.725; 6 -0.325,0.725; 7 0.325,0.725; 8 0.975,0.725
0402 = smd 0.85 x 0.9: 1 -0.58,0; 2 0.58,0
0603 = smd 1.1 x 1: 1 -0.85,0; 2 0.85,0
0805 = smd 0.8 x 1.2: 1 -0.9,0; 2 0.9,0
LED_SML-P11UTT86R = smd 0.5 x 0.6: A 0.45,0; C -0.45,0
BEADC0603X33N = smd 0.38 x 0.4: 1 -0.281,0; 2 0.281,0
FE05-1 = drill 0.813 long: 1 -5.08,0; 2 -2.54,0; 3 0,0; 4 2.54,0; 5 5.08,0
2X03 = drill 1.016 octagon: 1 -2.54,-1.27; 2 -2.54,1.27; 3 0,-1.27; 4 0,1.27; 5 2.54,-1.27; 6 2.54,1.27
B6B-ZR = drill 0.7: 1 9,-1.3; 2 7.5,-1.3; 3 6,-1.3; 4 4.5,-1.3; 5 3,-1.3; 6 1.5,-1.3
SON95P300X300X100-7N = smd 0.84 x 0.4: 1 -1.435,0.95; 2 -1.435,0; 3 -1.435,-0.95; 4 1.435,-0.95; 5 1.435,0; 6 1.435,0.95 | smd 1.625 x 2.365: 7 0,0
RESC1005X35N = smd 0.56 x 0.6: 1 -0.435,0; 2 0.435,0
LL3301FF065QJ = smd 2.1 x 1.4: 1 -3,2.25; 2 3,2.25; 3 -3,-2.25; 4 3,-2.25
DQD8_1P2X0P4 = smd 0.5 x 0.2: 1 -0.625,0.6; 2 -0.625,0.2; 3 -0.625,-0.2; 4 -0.625,-0.6; 5 0.625,-0.6; 6 0.625,-0.2; 7 0.625,0.2; 8 0.625,0.6 | smd 0.4 x 1.2: 9 0,0
PQFN50P450X300X100-16N = smd 0.35 x 0.59: 1 -1.5,1.165; 2 -1,1.165; 3 -0.5,1.165; 4 0,1.165; 5 0.5,1.165; 6 1,1.165; 7 1.5,1.165; 9 1.5,-1.165; 10 1,-1.165; 11 0.5,-1.165; 12 0,-1.165; 13 -0.5,-1.165; 14 -1,-1.165; 15 -1.5,-1.165 | smd 0.59 x 0.35: 8 1.915,0; 16 -1.915,0
QFP50P2200X2200X160-144N = smd 1.56 x 0.28: 1 -10.68,8.75; 2 -10.68,8.25; 3 -10.68,7.75; 4 -10.68,7.25; 5 -10.68,6.75; 6 -10.68,6.25; 7 -10.68,5.75; 8 -10.68,5.25; 9 -10.68,4.75; 10 -10.68,4.25; 11 -10.68,3.75; 12 -10.68,3.25; 13 -10.68,2.75; 14 -10.68,2.25; 15 -10.68,1.75; 16 -10.68,1.25; 17 -10.68,0.75; 18 -10.68,0.25; 19 -10.68,-0.25; 20 -10.68,-0.75; 21 -10.68,-1.25; 22 -10.68,-1.75; 23 -10.68,-2.25; 24 -10.68,-2.75; 25 -10.68,-3.25; 26 -10.68,-3.75; 27 -10.68,-4.25; 28 -10.68,-4.75; 29 -10.68,-5.25; 30 -10.68,-5.75; 31 -10.68,-6.25; 32 -10.68,-6.75; 33 -10.68,-7.25; 34 -10.68,-7.75; 35 -10.68,-8.25; 36 -10.68,-8.75; 73 10.68,-8.75; 74 10.68,-8.25; 75 10.68,-7.75; 76 10.68,-7.25; 77 10.68,-6.75; 78 10.68,-6.25; 79 10.68,-5.75; 80 10.68,-5.25; 81 10.68,-4.75; 82 10.68,-4.25; 83 10.68,-3.75; 84 10.68,-3.25; 85 10.68,-2.75; 86 10.68,-2.25; 87 10.68,-1.75; 88 10.68,-1.25; 89 10.68,-0.75; 90 10.68,-0.25; 91 10.68,0.25; 92 10.68,0.75; 93 10.68,1.25; 94 10.68,1.75; 95 10.68,2.25; 96 10.68,2.75; 97 10.68,3.25; 98 10.68,3.75; 99 10.68,4.25; 100 10.68,4.75; 101 10.68,5.25; 102 10.68,5.75; 103 10.68,6.25; 104 10.68,6.75; 105 10.68,7.25; 106 10.68,7.75; 107 10.68,8.25; 108 10.68,8.75 | smd 0.28 x 1.56: 37 -8.75,-10.68; 38 -8.25,-10.68; 39 -7.75,-10.68; 40 -7.25,-10.68; 41 -6.75,-10.68; 42 -6.25,-10.68; 43 -5.75,-10.68; 44 -5.25,-10.68; 45 -4.75,-10.68; 46 -4.25,-10.68; 47 -3.75,-10.68; 48 -3.25,-10.68; 49 -2.75,-10.68; 50 -2.25,-10.68; 51 -1.75,-10.68; 52 -1.25,-10.68; 53 -0.75,-10.68; 54 -0.25,-10.68; 55 0.25,-10.68; 56 0.75,-10.68; 57 1.25,-10.68; 58 1.75,-10.68; 59 2.25,-10.68; 60 2.75,-10.68; 61 3.25,-10.68; 62 3.75,-10.68; 63 4.25,-10.68; 64 4.75,-10.68; 65 5.25,-10.68; 66 5.75,-10.68; 67 6.25,-10.68; 68 6.75,-10.68; 69 7.25,-10.68; 70 7.75,-10.68; 71 8.25,-10.68; 72 8.75,-10.68; 109 8.75,10.68; 110 8.25,10.68; 111 7.75,10.68; 112 7.25,10.68; 113 6.75,10.68; 114 6.25,10.68; 115 5.75,10.68; 116 5.25,10.68; 117 4.75,10.68; 118 4.25,10.68; 119 3.75,10.68; 120 3.25,10.68; 121 2.75,10.68; 122 2.25,10.68; 123 1.75,10.68; 124 1.25,10.68; 125 0.75,10.68; 126 0.25,10.68; 127 -0.25,10.68; 128 -0.75,10.68; 129 -1.25,10.68; 130 -1.75,10.68; 131 -2.25,10.68; 132 -2.75,10.68; 133 -3.25,10.68; 134 -3.75,10.68; 135 -4.25,10.68; 136 -4.75,10.68; 137 -5.25,10.68; 138 -5.75,10.68; 139 -6.25,10.68; 140 -6.75,10.68; 141 -7.25,10.68; 142 -7.75,10.68; 143 -8.25,10.68; 144 -8.75,10.68
XDCR_LIS3MDLTR = smd 0.375 x 0.35: 1 -0.762,0.75; 2 -0.762,0.25; 3 -0.762,-0.25; 4 -0.762,-0.75; 7 0.762,-0.75; 8 0.762,-0.25; 9 0.762,0.25; 10 0.762,0.75 | smd 0.35 x 0.375: 5 -0.25,-0.762; 6 0.25,-0.762; 11 0.25,0.762; 12 -0.25,0.762
DIOM5226X223N = smd 2.4 x 1.55: 1 -2.1,0; 2 2.1,0
ECSTXO3225MV400TR = smd 1.3 x 1.1: 1 -1.15,-0.95; 2 1.15,-0.95; 3 1.15,0.95; 4 -1.15,0.95

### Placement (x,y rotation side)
BAROMETER  38.1,59.69 0 top
BAROMETER1  34.29,59.69 270 top
BAROMETER2  43.18,59.69 0 top
C1  38.1,55.88 0 top
C2  38.1,53.34 0 top
C3  3.81,3.81 180 top
C4  27.94,59.69 0 top
C5  41.91,53.34 0 top
C6  10.16,43.18 0 top
C7  8.89,48.26 90 top
C8  3.81,50.8 90 top
C9  6.35,45.72 270 top
C10  29.21,53.34 0 top
C11  27.94,62.23 0 top
C12  24.13,54.61 0 top
C13  41.91,55.88 0 top
C14  11.43,35.56 180 top
C15  10.16,22.86 0 top
C16  7.62,15.24 0 top
C17  10.16,19.05 0 top
C18  5.08,35.56 0 top
C19  7.62,39.37 0 top
C20  8.89,26.67 180 top
C21  8.89,31.75 180 top
C22  13.97,16.51 90 top
C23  19.05,40.64 0 top
C24  22.86,21.59 0 top
C25  30.48,21.59 0 top
C26  46.99,54.61 270 top
C27  15.24,12.7 0 top
C28  35.56,16.51 0 top
C29  43.18,21.59 0 top
C30  35.56,19.05 0 top
C31  48.26,15.24 90 top
C32  44.45,5.08 0 top
C33  35.56,21.59 0 top
C34  10.16,52.07 0 top
C35  13.97,26.67 0 top
C36  46.99,63.5 0 top
C37  48.26,26.67 90 top
D1  16.51,46.99 90 top
FL1  39.37,16.51 90 top
FL2  21.59,16.51 0 top
FL3  48.26,19.05 0 top
GPS  3.81,25.4 270 top
JP1  49.53,38.1 270 top
L1  6.35,41.91 0 top
L2  30.48,60.96 270 top
L3  44.45,55.88 90 top
L7  39.37,63.5 0 top
LIDAR  29.21,3.81 180 top
OP_FLOW  40.64,3.81 180 top
POWER_MODULE  3.81,63.5 0 top
R1  33.02,53.34 0 top
R2  33.02,55.88 0 top
R3  12.7,49.53 0 top
R4  33.02,63.5 0 top
R5  21.59,52.07 0 top
R6  35.56,50.8 0 top
R7  38.1,50.8 180 top
R8  26.67,16.51 0 top
R9  44.45,16.51 0 top
R11  8.89,10.16 90 top
R12  29.21,57.15 90 top
R13  49.53,54.61 0 top
R14  19.05,12.7 0 top
R15  43.18,63.5 90 top
R16  19.05,10.16 270 top
R17  41.91,16.51 0 top
R18  30.48,17.78 270 top
R19  24.13,17.78 180 top
R23  33.02,19.05 90 top
R24  46.99,22.86 270 top
RADIO  1.27,38.1 90 top
RC  17.78,3.81 180 top
S1  16.51,57.15 0 top
S2  6.35,57.15 0 top
U1  46.99,50.8 90 top
U2  35.56,12.7 0 top
U3  44.45,8.89 180 top
U4  26.67,12.7 0 top
U5  33.02,36.83 0 top
U9  16.51,50.8 0 top
U10  50.8,62.23 0 top
U11  15.24,21.59 0 top
U$1  24.13,60.96 90 top
Y1  3.81,10.16 0 top

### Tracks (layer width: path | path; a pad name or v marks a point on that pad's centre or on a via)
3V2
  Top 0.152: FL1.2 39.37,16.67 36.67,16.67 36.51,16.51 C28.2 36.35,16.51 35.56,15.72 | 35.56,15.72 34.92,15.08 34.92,13.97 U2.3 | C29.2 43.66,21.59 41.91,19.84 35.88,19.84 35.56,19.53 35.56,15.72
3V3  (via drill 0.35)
  Top 0.152: 40.8,63.5 v41.27,63.5 42.7,63.5 43.18,63.98 | 40.8,63.5 L7.2 | BAROMETER2.6 42.7,60.48 42.23,60.48 BAROMETER2.5 42.23,60.33 43.5,59.05 BAROMETER2.2 43.66,58.9 44.29,58.26 | L3.2 44.45,58.1 44.29,58.26 | 40.8,63.5 40.8,58.74 41.27,58.26 44.29,58.26 | U10.6 50.96,61.59 50.64,61.59 U10.5 50.48,61.44 50.48,57.47 | 50.48,57.47 50.48,54.93 50.16,54.61 R13.2 50.01,54.61 | 44.45,39.21 43.81,39.21 U5.95 43.66,39.05 v42.39,39.05 | 43.18,63.98 43.97,63.98 50.48,57.47 | 43.18,63.98 R15.2 | 5.71,32.23 5.71,34.13 4.29,35.56 C18.1 4.13,35.56 1.91,37.78 | 5.71,32.23 5.71,23.81 9.21,20.32 9.21,19.05 C17.1 | 9.84,27.46 9.84,31.75 C21.1 | 9.84,27.46 9.84,26.67 C20.1 | U5.30 22.38,30.96 22.38,30.64 U5.31 22.38,30.48 23.18,30.48 23.34,30.32 23.34,29.84 23.18,29.69 22.38,29.69 U5.33 22.23,29.53 21.59,29.53 19.05,26.99 19.05,23.5 17.62,22.07 | U11.6 15.4,20.95 15.08,20.95 U11.5 14.92,20.8 14.92,20.48 | 14.92,19.05 14.92,16.67 13.97,15.72 C22.1 | 14.92,19.05 14.92,20.48 | 14.92,20.48 11.59,20.48 9.84,22.23 9.84,22.38 9.37,22.86 C15.1 9.21,22.86 12.22,25.88 13.65,25.88 13.97,26.19 13.97,27.15 13.65,27.46 9.84,27.46 | 17.62,22.07 16.35,20.8 16.35,20.48 14.92,19.05 | U9.6 16.67,50.16 16.35,50.16 U9.5 16.19,50.01 16.19,49.85 15.88,49.53 | R3.2 v14.61,49.53 15.88,49.53 | 24.29,43.18 24.29,47.47 U5.144 24.29,47.62 24.77,47.62 U5.143 | 24.29,43.18 24.29,38.89 23.02,37.62 22.38,37.62 U5.17 | 24.29,43.18 22.38,43.18 U5.6 22.23,43.18 21.59,43.18 15.88,48.9 15.88,49.53 | 35.08,60.48 35.08,60.64 BAROMETER1.5 | 35.08,60.48 35.08,60.17 BAROMETER1.6 | BAROMETER.5 37.15,60.48 37.62,60.48 BAROMETER.6
  Top 0.152: BAROMETER.5 37.15,60.33 v37.78,59.69 38.42,59.05 BAROMETER.2 38.42,58.9 35.56,56.04 33.81,56.04 33.66,55.88 | 35.08,60.48 36.99,60.48 BAROMETER.5 | 33.66,55.88 33.66,53.34 | 33.66,53.34 30.8,50.48 30.8,47.62 U5.131 | 33.66,53.34 R1.2 | 33.66,55.88 R2.2 | C3.2 2.86,3.81 2.86,9.05 2.7,9.21 Y1.1 2.7,9.37 2.7,10.95 Y1.4 2.54,11.11 6.67,15.24 | S1.1 13.65,59.37 v16.51,59.37 19.37,59.37 S1.2 | v32.86,59.37 33.5,59.37 BAROMETER1.2 | L2.2 30.48,60.8 v29.69,60.8 29.69,62.71 29.37,63.02 28.26,63.02 27.94,62.71 27.94,58.58 28.73,57.78 29.21,57.78 R12.2 | v5.24,61.75 POWER_MODULE.4 | v23.65,55.56 23.65,54.61 C12.1 | v28.73,54.29 28.73,53.34 C10.1 | v37.47,54.29 37.47,53.34 C2.1 | v33.66,64.45 33.66,63.5 R4.2 | 25.4,27.15 25.4,26.19 U5.39 | v31.91,27.46 31.91,26.19 U5.52 | v36.83,27.46 36.83,26.19 U5.62 | v42.39,26.83 41.75,26.19 U5.72 | v45.09,33.66 43.81,33.66 U5.84 | v35.88,48.9 35.88,47.62 U5.121 | v45.09,45.56 43.81,45.56 U5.108 | 6.67,15.24 6.67,17.46 GPS.5 2.22,21.91 2.22,30.8 3.65,32.23 5.71,32.23 | 6.67,15.24 C16.1 | 17.62,22.07 18.26,21.43 18.57,21.43 23.02,25.88 23.02,26.19 23.97,27.15 25.4,27.15 | 25.4,27.15 v25.4,27.46 | 3.97,45.72 2.7,46.99 RADIO.1 2.7,47.15 3.81,47.15 C8.1 | 3.97,45.72 5.24,44.45 6.51,44.45 6.51,41.91 L1.2 | 3.97,45.72 5.87,45.72 6.35,46.2 C9.1
  pour Route15: 1.27,66.04 53.34,66.04 53.34,1.27 1.27,1.27
3V4
  Top 0.152: 21.91,18.41 21.91,19.84 23.65,21.59 C24.2 23.81,21.59 24.61,22.38 30.16,22.38 30.96,21.59 C25.2 | 21.91,18.41 21.91,16.51 FL2.2 | 21.91,18.41 26.04,14.29 26.04,13.97 U4.3
3V5
  Top 0.152: 45.09,7.14 45.09,5.24 45.24,5.08 C32.2 | 45.09,7.14 45.09,7.62 U3.3 | FL3.2 48.42,19.05 48.42,16.35 48.26,16.19 C31.2 48.26,16.03 49.05,15.24 49.05,7.46 48.74,7.14 45.09,7.14
5V
  Top 0.152: C6.1 9.53,43.18 8.89,43.81 C7.1 8.89,47.78 8.26,47.78 7.3,48.74 7.3,55.24 10.64,58.58 10.64,64.29 | POWER_MODULE.1 2.86,64.93 4.76,64.93 POWER_MODULE.6 5.4,64.29 10.64,64.29 | 10.64,64.29 18.73,64.29 24.13,58.9 U$1.1
BOOT0
  Top 0.152: U5.138 27.15,47.62 27.15,49.05 24.92,51.28 21.59,51.28 20.8,52.07 R5.1 20.64,52.07 20.64,53.66 19.53,54.77 S1.4 19.37,54.93 13.65,54.93 S1.3
CSB_ACCEL1  (via drill 0.35)
  Top 0.152: v25.56,12.38 25.56,11.59 U4.14 | v25.24,16.19 23.65,17.78 R19.2
  Bottom 0.152: v25.56,12.38 25.56,16.19 v25.24,16.19
CSB_ACCEL2
  Top 0.152: U3.14 45.4,10.16 45.4,16.03 44.93,16.51 R9.2
CSB_ACCEL3  (via drill 0.35)
  Top 0.152: v33.34,11.43 33.81,10.95 34.29,10.95 34.45,11.11 34.45,11.43 U2.14 | v33.5,49.21 35.08,50.8 R6.1
  Bottom 0.152: v33.34,11.43 33.34,23.34 35.08,23.34 40.01,28.26 42.23,28.26 43.02,29.05 43.02,41.91 38.89,41.91 35.88,44.93 30.32,44.93 30,45.24 28.57,45.24 28.42,45.4 28.42,48.26 32.54,48.26 v33.5,49.21
CSB_GYRO1
  Top 0.152: U4.5 27.15,13.97 27.15,16.51 R8.2
CSB_GYRO2  (via drill 0.35)
  Top 0.152: v43.97,8.57 43.97,7.78 U3.5 | v50.64,18.89 50.64,19.37 51.91,20.64 v51.91,30.16 | v44.61,47.31 41.12,50.8 R7.1
  Bottom 0.152: v43.97,8.57 43.97,13.02 44.77,13.02 v50.64,18.89 | v51.91,30.16 46.04,36.04 46.04,46.51 45.4,46.51 v44.61,47.31
CSB_GYRO3  (via drill 0.35)
  Top 0.152: v36.2,15.4 36.2,13.97 U2.5 | v45.09,30.32 44.45,30.96 43.81,30.96 U5.79
  Bottom 0.152: v36.2,15.4 36.2,23.97 38.73,23.97 v45.09,30.32
EXTI0
  Top 0.152: R14.2 U4.16
EXTI0_1
  Top 0.152: U2.12 35.56,11.27 34.61,10.32 30.64,10.32 29.37,11.59 29.37,17.3 29.84,17.78 31.59,17.78 32.38,18.57 32.38,19.05 33.02,19.68 R23.2
EXTI1  (via drill 0.35)
  Top 0.152: v47.15,8.89 U3.16 | v49.69,11.43 49.69,15.88 49.05,16.51 49.05,20.16 46.99,22.23 R24.2
  Bottom 0.152: v49.69,11.43 v47.15,8.89
EXTI2
  Top 0.152: U4.12 26.67,11.75 26.99,12.06 28.42,12.06 28.57,11.91 28.57,10.64 27.62,9.68 19.05,9.68 R16.2
EXTI3
  Top 0.152: U3.12 44.45,14.61 42.55,16.51 R17.2
EXTI4
  Top 0.152: U2.16 30,12.7 29.69,13.02 29.69,16.35 30.48,17.14 R18.2
GND  (via drill 0.35)
  Top 0.152: C35.1 11.43,26.67 10.32,25.56 8.57,25.56 | 8.57,25.56 7.94,26.19 7.94,26.67 | C14.2 7.94,35.56 | 7.94,35.56 6.67,35.56 | 6.67,35.56 C18.2 | 6.67,35.56 6.67,38.73 | 6.67,38.73 6.67,39.37 | 7.94,35.56 7.94,31.75 | 7.94,31.75 7.94,26.67 | 7.94,26.67 C20.2 | 7.94,31.75 C21.2 | U5.38 24.77,26.04 24.77,25.4 22.07,22.7 22.07,21.59 C24.1 21.91,21.59 14.29,13.97 | 14.29,13.97 14.29,12.7 C27.1 | 14.29,13.97 12.86,15.4 12.86,16.35 13.97,17.46 | 11.43,19.05 12.7,19.05 13.97,17.78 13.97,17.46 | 11.43,19.05 C17.2 | 13.97,17.46 C22.2 | 8.57,25.56 8.57,21.91 11.43,19.05 | U5.16 22.23,38.1 21.59,38.1 20,39.69 20,40.64 C23.2 19.53,40.64 17.3,42.86 10.95,42.86 10.64,43.18 C6.2 10.79,43.18 10.79,47.47 9.37,48.9 8.89,48.9 | 8.89,48.9 8.89,51.91 9.05,52.07 C34.1 9.37,52.07 9.37,54.77 S2.4 | 50.16,62.39 50.16,62.07 U10.3 | 50.16,62.39 50.48,62.71 50.48,62.87 U10.12 50.48,63.02 50.48,63.18 49.05,64.61 47.62,64.61 46.51,63.5 C36.1 44.93,63.5 43.34,65.09 39.37,65.09 35.72,61.44 | 50.16,62.39 U10.2 | C26.2 46.99,52.7 46.04,51.75 46.04,51.12 | 46.04,51.12 46.2,50.96 46.83,50.96 U1.9 | 42.55,55.88 42.55,53.34 | C13.2 42.55,55.88 | 38.73,55.88 38.73,53.34 C2.2 | 35.72,61.44 37.47,61.44 38.42,60.48 BAROMETER.7 38.58,60.33 39.21,59.69 39.21,59.05 BAROMETER.1 39.05,58.9 38.73,58.58 38.73,58.42 | 35.72,61.44 35.08,61.44 34.61,60.96 34.61,59.85 34.92,59.53 34.92,59.37 BAROMETER1.7 | 38.73,58.42 38.73,56.99 | 38.73,56.99 38.73,55.88 | 38.73,55.88 C1.2 | 42.55,55.88 42.39,55.88 41.27,56.99 38.73,56.99 | 46.04,51.12 39.05,51.12 37.78,52.39 37.31,52.39 36.51,53.18 36.51,56.2 38.73,58.42 | POWER_MODULE.7 POWER_MODULE.2 2.22,63.5 1.43,62.71 1.43,56.2 2.86,54.77
  Top 0.152: 2.86,54.77 3.02,54.93 3.33,54.93 S2.3 | 2.86,54.77 2.54,54.45 | 2.86,54.77 S2.3 | 28.57,60.01 28.57,62.23 C11.2 | 28.57,60.01 28.57,59.69 | C10.2 29.84,53.34 29.84,53.82 30.16,54.13 30.16,56.36 32.54,58.74 33.5,58.74 BAROMETER1.1 33.66,58.58 33.97,58.9 33.97,60.96 33.81,61.12 32.86,61.12 31.75,60.01 28.57,60.01 | 28.57,60.01 C4.2 28.57,59.69 | 34.77,19.05 v34.77,17.78 34.77,16.51 C28.1 | 34.77,19.05 34.77,20.48 | 34.77,20.48 34.77,21.59 C33.1 | 34.77,19.05 C30.1 | C29.1 37.94,21.59 36.83,20.48 34.77,20.48 | U4.4 26.67,13.65 26.99,13.34 27.46,13.34 27.62,13.49 27.62,13.81 U4.6 27.78,13.97 28.1,13.97 | 28.1,13.97 28.1,17.62 29.53,19.05 v29.53,20.32 29.53,21.59 C25.1 | 28.1,13.97 U4.7 | U5.51 31.27,26.19 31.27,27.15 31.11,27.3 31.11,27.62 31.59,28.1 v33.34,28.1 35.08,28.1 36.2,26.99 36.2,26.19 U5.61 | U5.83 43.66,33.18 42.86,33.18 v42.39,33.66 42.39,37.94 43.02,38.58 43.66,38.58 U5.94 | 4.76,6.19 4.76,9.21 4.92,9.37 Y1.2 | 4.76,6.19 4.76,3.81 C3.1 | 24.77,54.61 24.77,53.82 23.02,52.07 R5.2 | 14.61,21.75 14.61,21.43 U11.3 | 14.61,21.75 14.92,22.07 14.92,22.23 U11.12 | 14.61,21.75 U11.2 14.45,21.91 v13.49,21.91 12.38,21.91 11.43,22.86 C15.2 | 43.02,7.78 43.34,7.78 U3.6 | U3.4 44.45,7.46 44.13,7.14 43.81,7.14 43.5,7.46 | 43.5,7.46 43.34,7.62 U3.6 | 43.5,7.46 43.5,5.08 C32.1 | 43.5,7.46 U3.6 | BAROMETER2.7 43.66,60.33 44.29,59.69 44.29,59.05 BAROMETER2.1 44.29,58.9 v44.93,58.9 | 15.88,50.96 15.88,50.64 U9.3 | 15.88,50.96 16.19,51.28 16.19,51.44 U9.12 | 15.88,50.96 U9.2 15.72,51.12 v15.08,51.12 | 36.99,13.97 36.67,13.97 U2.6 | v35.56,14.76 U2.4 | v15.72,46.51 16.51,46.51 D1.C | v36.99,14.76 36.99,13.97
  Top 0.152: 36.99,13.97 U2.7 | v5.4,45.09 6.35,45.09 C9.2 | C16.2 v9.53,15.24 9.53,6.19 4.76,6.19 | v48.26,13.34 C31.1 | v47.15,27.62 48.26,27.62 C37.2 | v31.27,46.2 31.27,47.47 U5.130 | v36.2,46.2 36.2,47.47 U5.120 | v42.39,45.09 43.66,45.09 U5.107 | 43.02,7.78 43.02,9.21 42.86,9.37 42.23,9.37 39.21,6.35 39.21,5.24 OP_FLOW.6 | 43.02,7.78 U3.7 | v24.77,55.56 24.77,54.61 | 24.77,54.61 C12.2 | v28.57,58.74 28.57,59.69 | v42.55,52.39 42.55,53.34 | 42.55,53.34 C5.2 | v7.94,48.9 8.89,48.9 | 8.89,48.9 C7.2 | v6.67,40.48 6.67,39.37 | 6.67,39.37 C19.1 | S2.3 3.49,54.77 3.81,54.77 C8.2 3.81,51.28 3.33,50.8 3.17,50.8 1.75,49.37 1.75,38.73 6.67,38.73
  pour Route2: 1.27,66.04 53.34,66.04 53.34,1.27 1.27,1.27
GPIO1  (via drill 0.35)
  Top 0.152: v34.29,27.46 34.29,26.19 U5.57 | v35.56,24.77 35.56,23.81 33.97,22.23 33.97,16.03 v32.7,14.76 | v26.51,6.99 24.77,5.24 LIDAR.4
  Bottom 0.152: v34.29,27.46 35.56,26.19 v35.56,24.77 | v32.7,14.76 26.51,8.57 v26.51,6.99
GPIO_EXTI0  (via drill 0.35)
  Top 0.152: v18.41,13.65 18.41,12.7 R14.1 | v39.05,42.7 v18.41,22.07 | v39.21,45.09 39.21,45.72 39.53,46.04 39.53,46.51 39.37,46.67 39.37,47.47 U5.114
  Bottom 0.152: v18.41,22.07 v18.41,13.65 | v39.05,42.7 39.05,45.09 v39.21,45.09
GPIO_EXTI00
  Top 0.152: R23.1 33.02,18.57 33.5,19.05 33.66,19.05 33.66,23.5 33.02,24.13 33.02,24.77 33.66,25.4 33.66,26.04 U5.56
GPIO_EXTI1  (via drill 0.35)
  Top 0.152: R24.1 46.99,23.5 47.31,23.5 49.05,25.24 49.05,26.19 48.42,26.83 43.34,26.83 41.91,28.26 v41.91,28.89 41.75,29.05 41.75,39.37 42.07,39.69 v42.07,42.55 | v38.89,46.2 38.89,47.47 U5.115
  Bottom 0.152: v41.91,28.89 41.75,28.73 5.56,28.73 GPS.1 | v38.89,46.2 42.07,43.02 v42.07,42.55
GPIO_EXTI2  (via drill 0.35)
  Top 0.152: v7.3,34.61 7.3,22.7 10.16,19.84 10.16,18.57 10.79,17.94 10.79,14.92 14.92,10.79 19.05,10.79 R16.1 | v34.61,40.32 35.24,40.96 35.4,40.96 38.26,43.81 38.26,47.47 U5.116
  Bottom 0.152: v7.3,34.61 13.02,40.32 v34.61,40.32
GPIO_EXTI3  (via drill 0.35)
  Top 0.152: v41.27,19.21 41.27,16.51 R17.1 | v35.24,41.59 35.24,43.02 37.78,45.56 37.78,47.47 U5.117
GPIO_EXTI4  (via drill 0.35)
  Top 0.152: R18.1 30.48,18.89 32.86,21.27 32.86,23.02 31.11,24.77 v30.8,24.77 | v30.8,28.1 30.8,33.5 v35.88,38.58 | v35.72,44.29 35.72,44.93 37.15,46.35 37.15,47.47 U5.118
  Bottom 0.152: v30.8,28.1 v30.8,24.77 | v35.88,38.58 35.88,44.29 v35.72,44.29
I2C1_SCL  (via drill 0.35)
  Top 0.152: 32.38,53.34 31.75,53.98 31.75,56.36 32.7,57.31 34.29,57.31 35.88,58.9 36.99,58.9 BAROMETER.4 | v26.51,48.9 26.67,48.74 26.67,47.62 U5.139 | v28.89,49.21 28.89,49.85 32.38,53.34 | 32.38,53.34 R1.1
  Bottom 0.152: v26.51,48.9 26.83,49.21 v28.89,49.21
I2C1_SDA  (via drill 0.35)
  Top 0.152: 32.38,55.88 33.02,56.52 35.24,56.52 37.62,58.9 BAROMETER.3 | v25.88,49.53 25.88,48.74 26.19,48.42 26.19,47.62 U5.140 | 32.38,55.88 v32.38,54.29 | 32.38,55.88 R2.1
  Bottom 0.152: v25.88,49.53 28.42,49.53 32.38,53.5 v32.38,54.29
I2C2_SCL
  Top 0.152: 28.26,57.47 26.35,59.37 26.35,62.87 27.15,63.66 32.23,63.66 32.38,63.5 R4.1 | 28.26,57.47 28.57,57.15 29.84,57.15 29.84,57.63 32.86,60.64 33.5,60.64 BAROMETER1.4 | 28.26,57.47 13.97,57.47 10.16,53.66 10.16,50.32 14.61,45.88 16.03,45.88 20.8,41.12 22.23,41.12 U5.10
I2C2_SDA  (via drill 0.35)
  Top 0.152: BAROMETER1.3 33.5,60.01 32.7,60.01 30.16,57.47 30.16,56.99 29.84,56.67 29.21,56.67 R12.1 29.21,56.52 26.83,54.13 v26.83,50.16 | v23.65,41.27 23.02,40.64 22.38,40.64 U5.11
  Bottom 0.152: v23.65,41.27 23.65,45.09 23.81,45.09 25.24,46.51 25.24,50.16 v26.83,50.16
I2C3_SCL  (via drill 0.35)
  Top 0.152: v41.43,58.9 42.07,58.9 BAROMETER2.4 | v48.1,55.4 48.9,54.61 R13.1 49.05,54.61 49.05,53.98 51.12,51.91 v51.12,50.16 | 44.45,41.59 43.81,41.59 U5.100 44.45,41.59 | v48.26,45.4 44.45,41.59
  Bottom 0.152: v41.43,58.9 44.93,55.4 v48.1,55.4 | v48.26,45.4 50.8,47.94 50.8,49.85 v51.12,50.16
I2C3_SDA
  Top 0.152: 42.86,62.55 43.18,62.87 R15.1 42.86,62.55 | 42.86,62.55 41.75,61.44 41.75,60.01 42.7,59.05 BAROMETER2.3 | 44.45,41.12 43.81,41.12 U5.99 44.45,41.12 | 42.86,62.55 49.53,55.88 49.53,53.98 52.39,51.12 52.39,40.8 51.28,39.69 47.78,39.69 46.35,41.12 44.45,41.12
I2C4_SCL  (via drill 0.35)
  Top 0.152: v50.01,27.62 45.56,32.07 43.81,32.07 U5.81
  Bottom 0.152: v50.01,27.62 50.01,18.73 48.9,18.73 42.23,12.06 35.08,12.06 28.89,5.87 22.38,5.87 21.75,5.24 LIDAR.2
I2C4_SDA  (via drill 0.35)
  Top 0.152: v33.97,39.69 27.78,45.88 27.78,47.47 U5.137 | v42.39,32.7 43.66,32.7 U5.82 | v5.08,31.59 5.4,31.27 5.4,21.59 10.48,16.51 10.48,14.76 16.35,8.89 19.05,8.89 22.7,5.24 23.18,5.24 LIDAR.3
  Bottom 0.152: v42.39,32.7 40.96,32.7 v33.97,39.69 13.18,39.69 v5.08,31.59
IMU_INT3
  Top 0.152: U3.13 45.09,10 45.09,9.68 45.24,9.53 45.72,9.53 45.72,8.26 46.04,7.94 U3.1
N$1
  Top 0.152: R11.1 8.89,9.68 6.35,9.68 5.08,10.95 Y1.3
N$2
  Top 0.152: C13.1 41.12,55.88 41.27,55.72 41.27,53.34 C5.1 41.43,53.34 41.43,52.7 42.39,51.75 42.7,51.75 44.45,53.5 L3.1 44.45,55.72 44.77,55.72 45.56,56.52 45.56,59.05 44.29,60.33 BAROMETER2.8
N$3
  Top 0.152: 27.15,62.23 27.3,62.07 27.3,59.69 C4.1 | 31.43,61.44 30.64,61.44 30.48,61.28 L2.1 | 31.43,61.44 33.97,61.44 34.29,61.12 34.29,59.37 34.92,58.74 BAROMETER1.8 | 27.15,62.23 27.62,62.71 27.62,62.87 28.1,63.34 29.53,63.34 31.43,61.44 | 27.15,62.23 C11.1
N$4
  Top 0.152: U9.4 15.72,50.16 13.02,50.16 11.11,52.07 C34.2
N$5
  Top 0.152: D1.A 16.51,47.47 14.13,47.47 12.06,49.53 R3.1
N$6  (via drill 0.35)
  Top 0.152: L7.1 39.21,63.5 39.21,60.48 BAROMETER.8 39.21,60.33 39.53,60.01 v39.53,58.42 | 38.1,54.45 37.62,54.93 37.62,55.88 C1.1 | 38.1,54.45 38.1,52.7 39.37,51.44 43.02,51.44 46.99,55.4 C26.1 | 38.1,54.45 v38.1,56.99
  Bottom 0.152: v38.1,56.99 v39.53,58.42
N$7
  Top 0.152: U11.4 14.45,20.95 11.59,20.95 10.16,22.38 10.16,23.34 12.38,25.56 13.81,25.56 14.92,26.67 C35.2
N$8
  Top 0.152: FL2.1 20,16.51 19.05,15.56 | 19.05,15.56 16.19,12.7 C27.2 | 19.05,15.56 19.05,12.06 20.48,10.64 26.51,10.64 27.15,11.27 27.15,11.43 U4.11
N$9
  Top 0.152: 39.37,16.03 39.37,15.4 36.2,12.22 36.2,11.59 U2.11 | 39.37,16.03 FL1.1 | C30.2 37.78,19.05 39.85,16.99 39.85,16.51 39.37,16.03
N$10
  Top 0.152: 44.61,22.38 45.88,21.11 | 45.88,21.11 47.94,19.05 FL3.1 | 37.31,22.38 36.51,21.59 C33.2 | 45.88,21.11 41.91,17.14 41.91,15.88 42.39,15.88 43.81,14.45 43.81,10.16 U3.11
N$11
  Top 0.152: U10.4 50.01,61.59 49.69,61.59 47.78,63.5 C36.2
N$12
  Top 0.152: C37.1 48.26,25.72 42.55,25.72 41.91,25.08 41.59,25.08 41.27,25.4 41.27,26.04 U5.71 41.27,26.19 41.27,42.86 42.86,44.45 43.66,44.45 U5.106
N$13
  Top 0.152: R6.2 35.88,50.8 35.88,49.85 34.77,48.74 34.77,47.62 U5.123
N$14  (via drill 0.35)
  Top 0.152: v36.83,50.8 R7.2 | v32.23,45.56 32.86,45.56 33.81,46.51 34.92,46.51 35.24,46.83 35.24,47.47 U5.122
  Bottom 0.152: v36.83,50.8 33.5,47.47 29.84,47.47 28.73,46.35 28.73,45.56 v32.23,45.56
N$15  (via drill 0.35)
  Top 0.152: v26.19,19.37 24.61,17.78 R19.1 | v33.66,24.29 34.77,25.4 34.77,26.04 U5.58
  Bottom 0.152: v26.19,19.37 31.11,24.29 v33.66,24.29
N$16  (via drill 0.35)
  Top 0.152: v27.78,19.37 26.35,17.94 26.35,16.51 R8.1 | v34.61,24.45 34.61,24.77 35.24,25.4 35.24,26.04 U5.59
  Bottom 0.152: v27.78,19.37 32.07,23.65 33.81,23.65 v34.61,24.45
N$17  (via drill 0.35)
  Top 0.152: v43.97,17.46 43.97,16.51 R9.1 | v38.26,23.02 35.88,25.4 35.88,26.04 U5.60
  Bottom 0.152: v43.97,17.46 38.42,23.02 v38.26,23.02
N$19
  Bottom 0.152: RC.6 16.19,5.08 15.88,5.08 15.08,4.29 8.41,4.29 1.59,11.11 1.59,38.58 2.54,39.53 RADIO.6
N$20
  Top 0.152: U4.13 26.04,11.75 26.35,12.06 26.35,12.38 25.08,13.65 U4.1
N$23
  Top 0.152: U2.13 34.92,11.75 35.24,12.06 35.24,12.7 34.61,13.34 33.97,13.34 33.97,13.65 U2.1
NRST  (via drill 0.35)
  Top 0.152: POWER_MODULE.3 2.38,60.48 3.33,59.53 S2.1 3.49,59.37 6.99,59.37 | 6.99,59.37 9.21,59.37 S2.2 | v48.1,49.69 47.62,50.16 U1.4 | v46.51,47.62 46.2,47.62 44.45,45.88 40.96,45.88 28.73,33.66 22.38,33.66 U5.25 22.23,33.66 20.95,33.66 18.26,36.35 18.26,40.64 C23.1 10.95,40.64 6.99,44.61 6.99,59.37
  Bottom 0.152: v48.1,49.69 46.51,49.69 v46.51,47.62
NRST_O  (via drill 0.35)
  Top 0.152: v47.94,52.07 47.62,52.07 47.62,51.44 U1.5 47.62,51.28 48.74,51.28 v51.44,48.58
  Route15 0.152: 53.18,35.56 53.34,35.72 53.34,46.67 v51.44,48.58
  Bottom 0.152: JP1.6 50.8,36.51 51.75,37.47 51.75,48.26 v51.44,48.58
SPI1_MISO  (via drill 0.35)
  Top 0.152: v24.45,11.59 25.08,11.59 U4.15 | v26.83,24.77 26.83,26.04 U5.42
  Bottom 0.152: v24.45,11.59 24.45,24.77 v26.83,24.77
SPI1_MOSI  (via drill 0.35)
  Top 0.152: v27.78,10.64 28.1,10.95 28.1,11.43 U4.9 | v32.23,22.86 31.91,22.86 29.69,25.08 27.62,25.08 27.3,25.4 27.3,26.04 U5.43
  Bottom 0.152: v27.78,10.64 32.23,15.08 v32.23,22.86
SPI1_SCK
  Top 0.152: U4.8 28.73,12.7 28.73,17.78 31.75,20.8 31.91,20.8 32.07,20.95 32.07,22.23 30.16,24.13 26.67,24.13 26.19,24.61 26.19,26.04 U5.41
SPI2_MISO  (via drill 0.35)
  Top 0.152: v47.15,18.89 46.04,17.78 46.04,10.16 U3.15 | v49.37,21.11 49.37,27.78 47.94,29.21 43.81,29.21 U5.75
  Bottom 0.152: v49.37,21.11 v47.15,18.89
SPI2_MOSI  (via drill 0.35)
  Top 0.152: v43.02,14.13 43.02,10.16 U3.9 | v45.88,27.46 43.18,27.46 42.7,27.94 42.7,29.21 43.02,29.53 43.66,29.53 U5.76
  Bottom 0.152: v43.02,14.13 43.02,14.61 45.88,17.46 v45.88,27.46
SPI2_SCK  (via drill 0.35)
  Top 0.152: v52.07,10.32 52.07,10 46.35,4.29 43.02,4.29 42.55,4.76 U3.8 | v47.78,28.57 43.81,28.57 U5.74
  Bottom 0.152: v52.07,10.32 52.07,28.57 v47.78,28.57
SPI3_MISO  (via drill 0.35)
  Top 0.152: v34.61,12.38 34.13,11.91 34.13,11.59 U2.15 | v46.67,36.2 v46.67,32.23 | v43.18,47.94 42.55,47.94 41.91,48.58 40.64,48.58 40.32,48.26 40.32,47.62 U5.112
  Bottom 0.152: v34.61,12.38 34.92,12.7 42.39,12.7 46.51,16.83 46.51,32.23 v46.67,32.23 | v46.67,36.2 46.67,46.83 45.88,46.83 44.77,47.94 v43.18,47.94
SPI3_MOSI  (via drill 0.35)
  Top 0.152: v37.78,11.43 37.15,11.43 U2.9 | v52.07,9.21 v50.8,7.94 | v41.12,49.53 39.85,48.26 39.85,47.62 U5.113
  Bottom 0.152: v37.78,11.43 41.27,7.94 v50.8,7.94 | v52.07,9.21 52.7,9.84 52.7,50.8 42.39,50.8 v41.12,49.53
SPI3_SCK  (via drill 0.35)
  Top 0.152: v38.26,13.34 37.62,12.7 U2.8 | v40.48,46.2 40.48,46.51 40.64,46.67 40.64,47.47 U5.111
  Bottom 0.152: v38.26,13.34 41.75,16.83 44.13,16.83 45.24,17.94 45.24,29.69 45.72,30.16 45.72,46.2 v40.48,46.2
SPI4_CS
  Top 0.152: U9.10 17.3,51.44 17.62,51.44 21.27,47.78 21.27,44.93 21.59,44.61 22.23,44.61 U5.3
SPI4_MISO  (via drill 0.35)
  Top 0.152: v20.64,49.21 17.94,51.91 16.99,51.91 16.83,51.75 16.83,51.59 U9.11 | v23.65,45.72 23.65,44.77 23.02,44.13 22.38,44.13 U5.4
  Bottom 0.152: v20.64,49.21 20.64,45.72 v23.65,45.72
SPI4_MOSI
  Top 0.152: U9.9 17.3,50.96 17.46,50.96 20.95,47.47 20.95,44.29 21.59,43.66 22.23,43.66 U5.5
SPI4_SCK
  Top 0.152: U9.1 15.88,51.59 15.88,51.91 16.19,52.23 18.41,52.23 22.23,48.42 22.23,45.56 U5.1
SPI5_CS  (via drill 0.35)
  Top 0.152: v17.3,29.37 17.3,26.83 16.03,25.56 16.03,22.38 U11.10 | v23.65,35.72 23.65,36.51 23.18,36.99 22.38,36.99 U5.18
  Bottom 0.152: v23.65,35.72 v17.3,29.37
SPI5_MISO  (via drill 0.35)
  Top 0.152: v16.67,30 16.67,26.67 15.56,25.56 15.56,22.38 U11.11 | v20.8,34.61 20.8,35.24 21.59,36.04 22.23,36.04 U5.20
  Bottom 0.152: v16.67,30 20.8,34.13 v20.8,34.61
SPI5_MOSI  (via drill 0.35)
  Top 0.152: v18.73,29.37 18.73,24.45 16.19,21.91 16.03,21.91 U11.9 | v23.65,34.29 23.65,34.92 23.02,35.56 22.38,35.56 U5.21
  Bottom 0.152: v23.65,34.29 v18.73,29.37
SPI5_SCK  (via drill 0.35)
  Top 0.152: v16.03,30.8 16.03,26.51 14.61,25.08 14.61,22.38 U11.1 | v20.16,35.24 21.43,36.51 22.23,36.51 U5.19
  Bottom 0.152: v16.03,30.8 20.16,34.92 v20.16,35.24
SPI6_CS
  Top 0.152: U10.10 51.59,62.87 52.07,62.87 52.07,51.91 52.7,51.28 52.7,39.05 | U5.93 43.81,38.1 44.45,38.1 45.09,38.73 45.09,39.05 52.7,39.05 | 52.7,39.05 52.7,9.05 47.62,3.97 39.21,3.97 38.1,5.08 37.78,5.08 OP_FLOW.5
SPI6_MISO  (via drill 0.35)
  Top 0.152: v50.96,63.66 50.96,63.02 U10.11 | v35.88,55.56 35.88,52.39 32.86,49.37 32.86,47.62 U5.127
  Bottom 0.152: 50.16,62.87 46.83,59.53 39.85,59.53 v35.88,55.56 | 50.16,62.87 v50.96,63.66 | 50.16,62.87 53.34,62.87 53.34,9.21 48.42,4.29 35.56,4.29 34.77,5.08 OP_FLOW.3
SPI6_MOSI  (via drill 0.35)
  Top 0.152: v50.8,62.23 50.96,62.39 51.44,62.39 U10.9 | v31.75,48.9 31.75,47.62 U5.129
  Bottom 0.152: v50.8,62.23 50.8,58.9 50.32,58.9 49.05,57.63 49.05,51.44 | 49.05,51.44 34.29,51.44 v31.75,48.9 | 49.05,51.44 53.02,51.44 53.02,9.37 50.96,7.3 38.26,7.3 36.2,5.24 OP_FLOW.4
SPI6_SCK  (via drill 0.35)
  Top 0.152: v49.37,62.87 50.01,62.87 U10.1 | v34.92,55.4 34.92,51.91 32.38,49.37 32.38,47.62 U5.128 | v52.07,63.5 53.02,62.55 53.02,8.89 47.78,3.65 34.92,3.65 33.5,5.08 33.18,5.08 OP_FLOW.2
  Bottom 0.152: v34.92,55.4 39.37,59.85 46.35,59.85 v49.37,62.87 50.8,64.29 51.28,64.29 v52.07,63.5
SWCLK
  Top 0.152: U5.109 41.75,47.47 42.55,46.67 44.77,46.67 45.24,47.15 45.24,47.94 46.83,49.53 46.83,50.16 U1.2
SWDIO  (via drill 0.35)
  Top 0.152: U5.105 43.81,44.13 44.45,44.13 47.31,46.99 v47.31,47.15 | v47.15,49.05 47.15,50.16 U1.3
  Bottom 0.152: v47.15,49.05 47.31,48.9 v47.31,47.15
SWO  (via drill 0.35)
  Top 0.152: v45.72,50.16 46.35,50.16 U1.1 | v30.32,46.2 29.84,46.67 29.84,47.47 U5.133
  Bottom 0.152: v45.72,50.16 44.13,48.58 36.67,48.58 34.92,46.83 30.96,46.83 v30.32,46.2
SWO_O  (via drill 0.35)
  Top 0.152: U1.8 46.35,51.44 46.35,51.59 47.78,53.02 v48.1,53.02 48.1,52.7 | 50.48,50.32 50.48,50.01 51.28,49.21 51.59,49.21 52.07,48.74 52.07,44.45
  Route2 0.152: 48.1,52.7 v48.1,53.02
UART4_RX  (via drill 0.35)
  Top 0.152: v45.09,43.02 43.81,43.02 U5.103 | v45.09,37.78 47.31,37.78 47.31,37.47 47.62,37.15 50.8,37.15 JP1.4
  Route2 0.152: 45.09,42.39 v45.09,43.02 | JP1.4 50.64,37.94
  Bottom 0.152: v45.09,37.78 v45.09,43.02
UART4_TX  (via drill 0.35)
  Top 0.152: v47.31,45.24 45.72,43.66 43.81,43.66 U5.104
  Bottom 0.152: v47.31,45.24 47.31,44.13 JP1.2
UART5_RX  (via drill 0.35)
  Top 0.152: v29.84,44.61 28.73,45.72 28.73,47.47 U5.135
  Bottom 0.152: v29.84,44.61 25.88,40.64 12.06,40.64 2.22,30.8 2.22,11.59 5.4,11.59 11.75,5.24 RC.3
UART5_TX  (via drill 0.35)
  Top 0.152: v28.26,50.16 28.26,47.62 U5.136
  Bottom 0.152: v28.26,50.16 27.62,50.8 21.43,50.8 1.91,31.27 1.91,11.27 4.13,11.27 10.16,5.24 RC.2
UART8_RX  (via drill 0.35)
  Top 0.152: v25.88,46.2 25.88,47.47 U5.141
  Bottom 0.152: v25.88,46.2 28.26,48.58 29.05,48.58 33.02,52.55 33.02,54.45 32.54,54.93 9.21,54.93 1.75,47.47 1.75,44.93 2.54,44.13 RADIO.3
UART8_TX  (via drill 0.35)
  Top 0.152: v15.72,52.55 18.57,52.55 20.64,50.48 25.24,50.48 25.24,47.62 U5.142
  Bottom 0.152: v15.72,52.55 9.53,52.55 2.7,45.72 RADIO.2
USART2_RX  (via drill 0.35)
  Top 0.152: v23.65,26.04 24.29,26.04 U5.37
  Bottom 0.152: v23.65,26.04 23.02,25.4 GPS.3
USART2_TX  (via drill 0.35)
  Top 0.152: v20.95,28.1 22.23,28.1 U5.36
  Bottom 0.152: v20.95,28.1 20.8,27.94 GPS.2
VREF
  Top 0.152: U5.32 22.23,30.16 17.78,30.16 12.38,35.56 C14.1 12.22,35.56 8.41,39.37 C19.2 8.57,39.37 6.83,41.12 6.19,41.12 6.19,41.91 L1.1
XSHUT  (via drill 0.35)
  Top 0.152: v20.32,24.77 23.65,28.1 23.65,31.91 23.02,32.54 22.38,32.54 U5.27
  Bottom 0.152: v20.32,24.77 19.37,23.81 19.37,4.76 19.84,4.29 26.19,4.29 26.19,5.08 LIDAR.5

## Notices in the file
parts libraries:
SparkFun-Capacitors: Licensing: Creative Commons ShareAlike 4.0 International - https://creativecommons.org/licenses/by-sa/4.0
